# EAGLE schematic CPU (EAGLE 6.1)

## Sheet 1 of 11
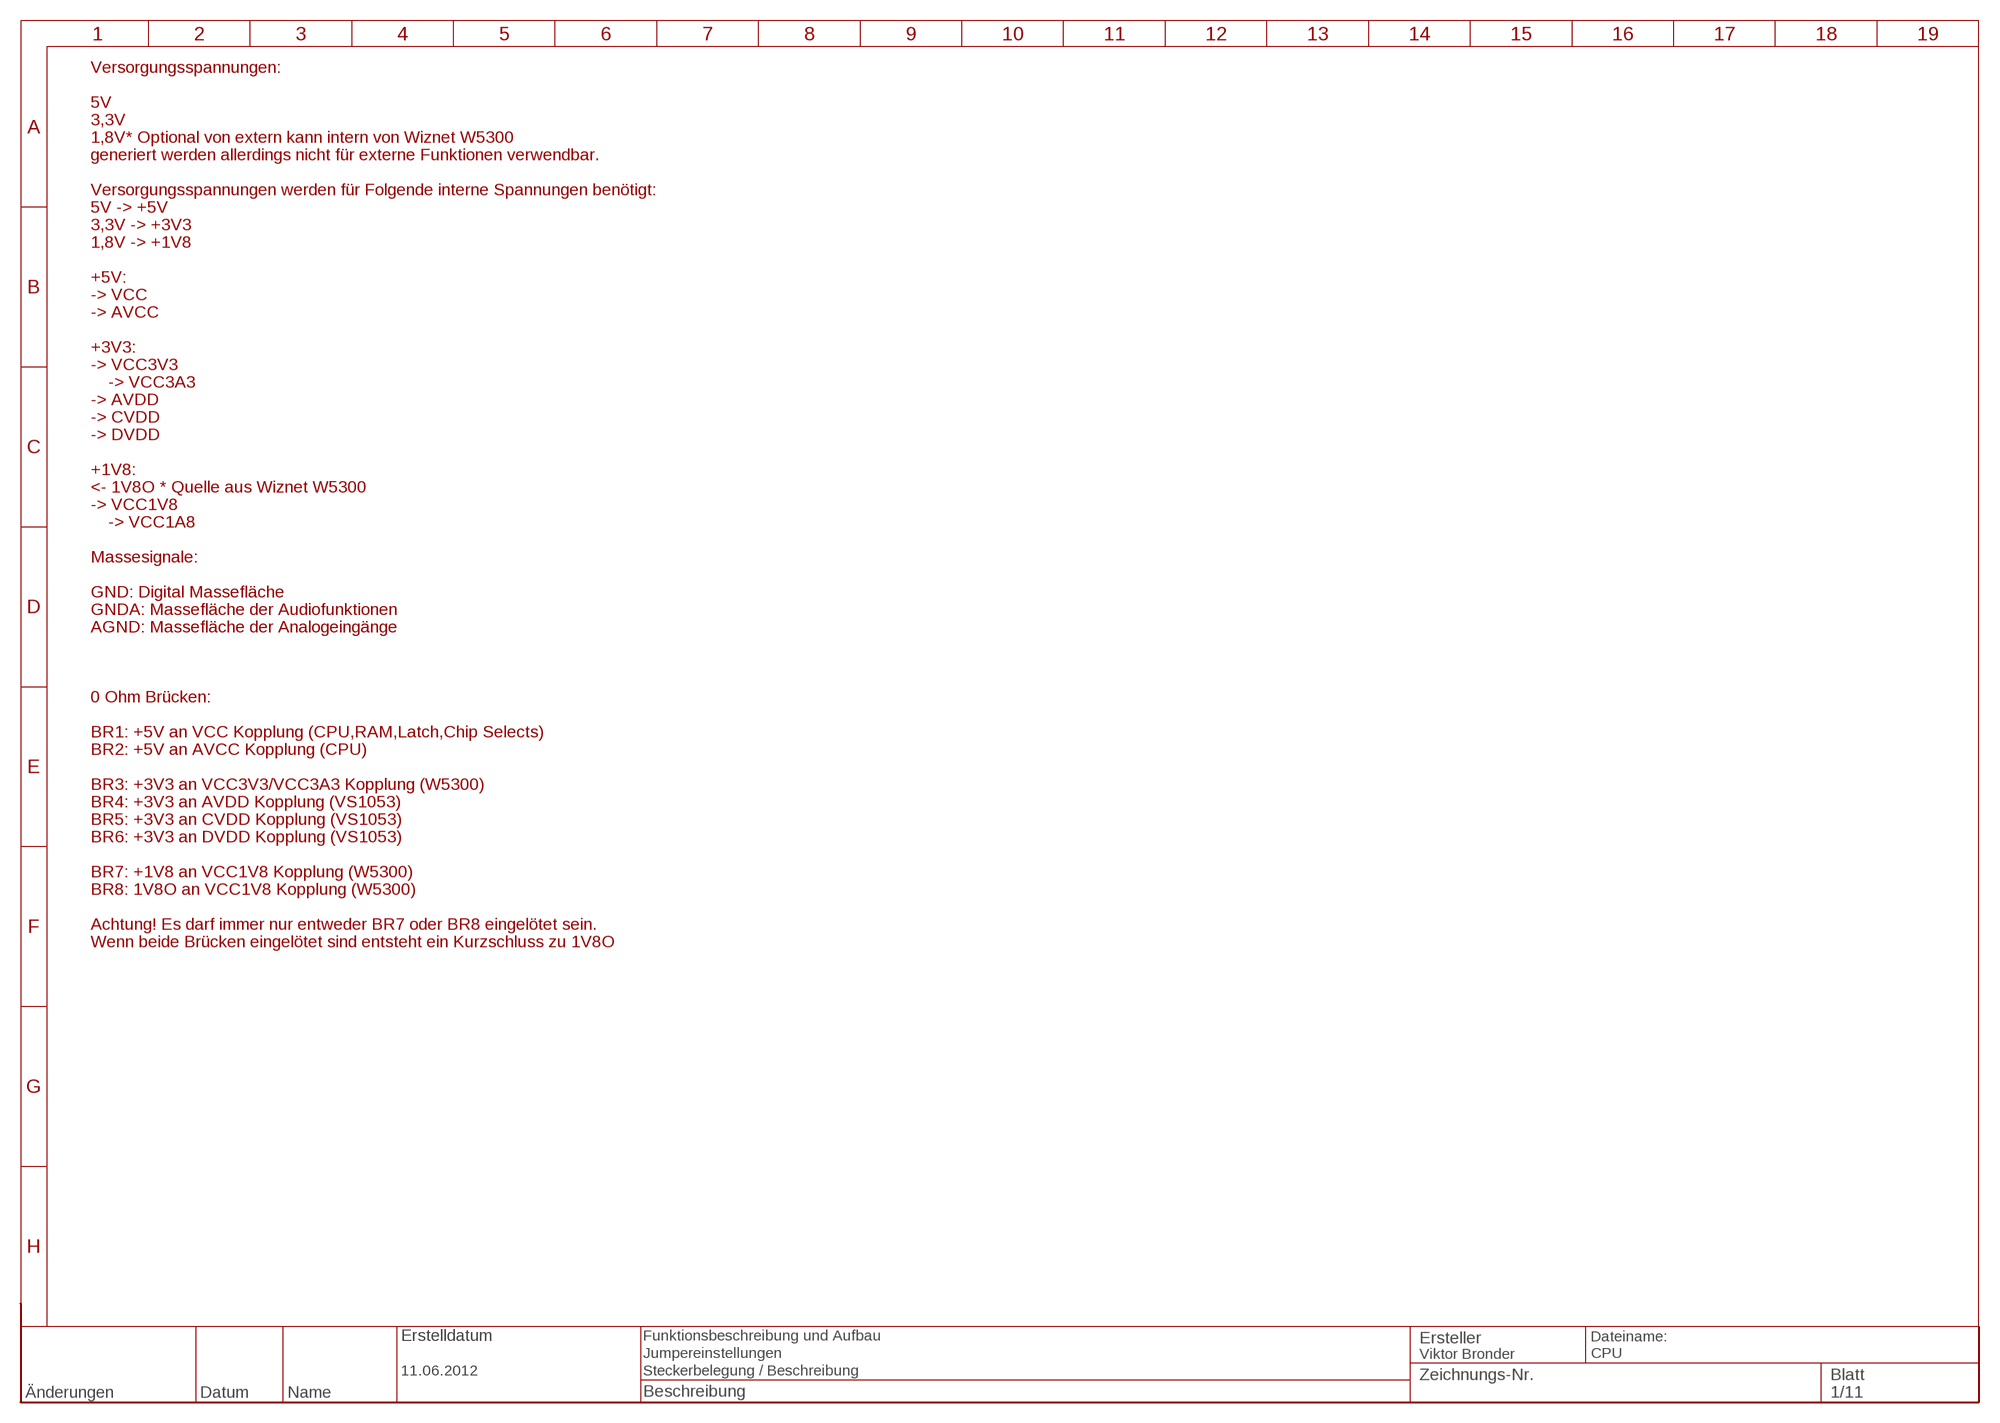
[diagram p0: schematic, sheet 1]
RAHMEN1 (RAHMEN_A4_8Z-19S): BESCHREIBUNG1: Funktionsbeschreibung und Aufbau; BESCHREIBUNG2: Jumpereinstellungen; BESCHREIBUNG3: Steckerbelegung / Beschreibung; ERSTELLDATUM: 11.06.2012; ERSTELLER: Viktor Bronder

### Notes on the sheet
- Versorgungsspannungen:
- 5V
- 3,3V
- 1,8V* Optional von extern kann intern von Wiznet W5300
- generiert werden allerdings nicht für externe Funktionen verwendbar.
- Versorgungsspannungen werden für Folgende interne Spannungen benötigt:
- 5V -> +5V
- 3,3V -> +3V3
- 1,8V -> +1V8
- +5V:
- -> VCC
- -> AVCC
- +3V3:
- -> VCC3V3
- -> VCC3A3
- -> AVDD
- -> CVDD
- -> DVDD
- +1V8:
- <- 1V8O * Quelle aus Wiznet W5300
- -> VCC1V8
- -> VCC1A8
- Massesignale:
- GND: Digital Massefläche
- GNDA: Massefläche der Audiofunktionen
- AGND: Massefläche der Analogeingänge
- 0 Ohm Brücken:
- BR1: +5V an VCC Kopplung (CPU,RAM,Latch,Chip Selects)
- BR2: +5V an AVCC Kopplung (CPU)
- BR3: +3V3 an VCC3V3/VCC3A3 Kopplung (W5300)
- BR4: +3V3 an AVDD Kopplung (VS1053)
- BR5: +3V3 an CVDD Kopplung (VS1053)
- BR6: +3V3 an DVDD Kopplung (VS1053)
- BR7: +1V8 an VCC1V8 Kopplung (W5300)
- BR8: 1V8O an VCC1V8 Kopplung (W5300)
- Achtung! Es darf immer nur entweder BR7 oder BR8 eingelötet sein.
- Wenn beide Brücken eingelötet sind entsteht ein Kurzschluss zu 1V8O

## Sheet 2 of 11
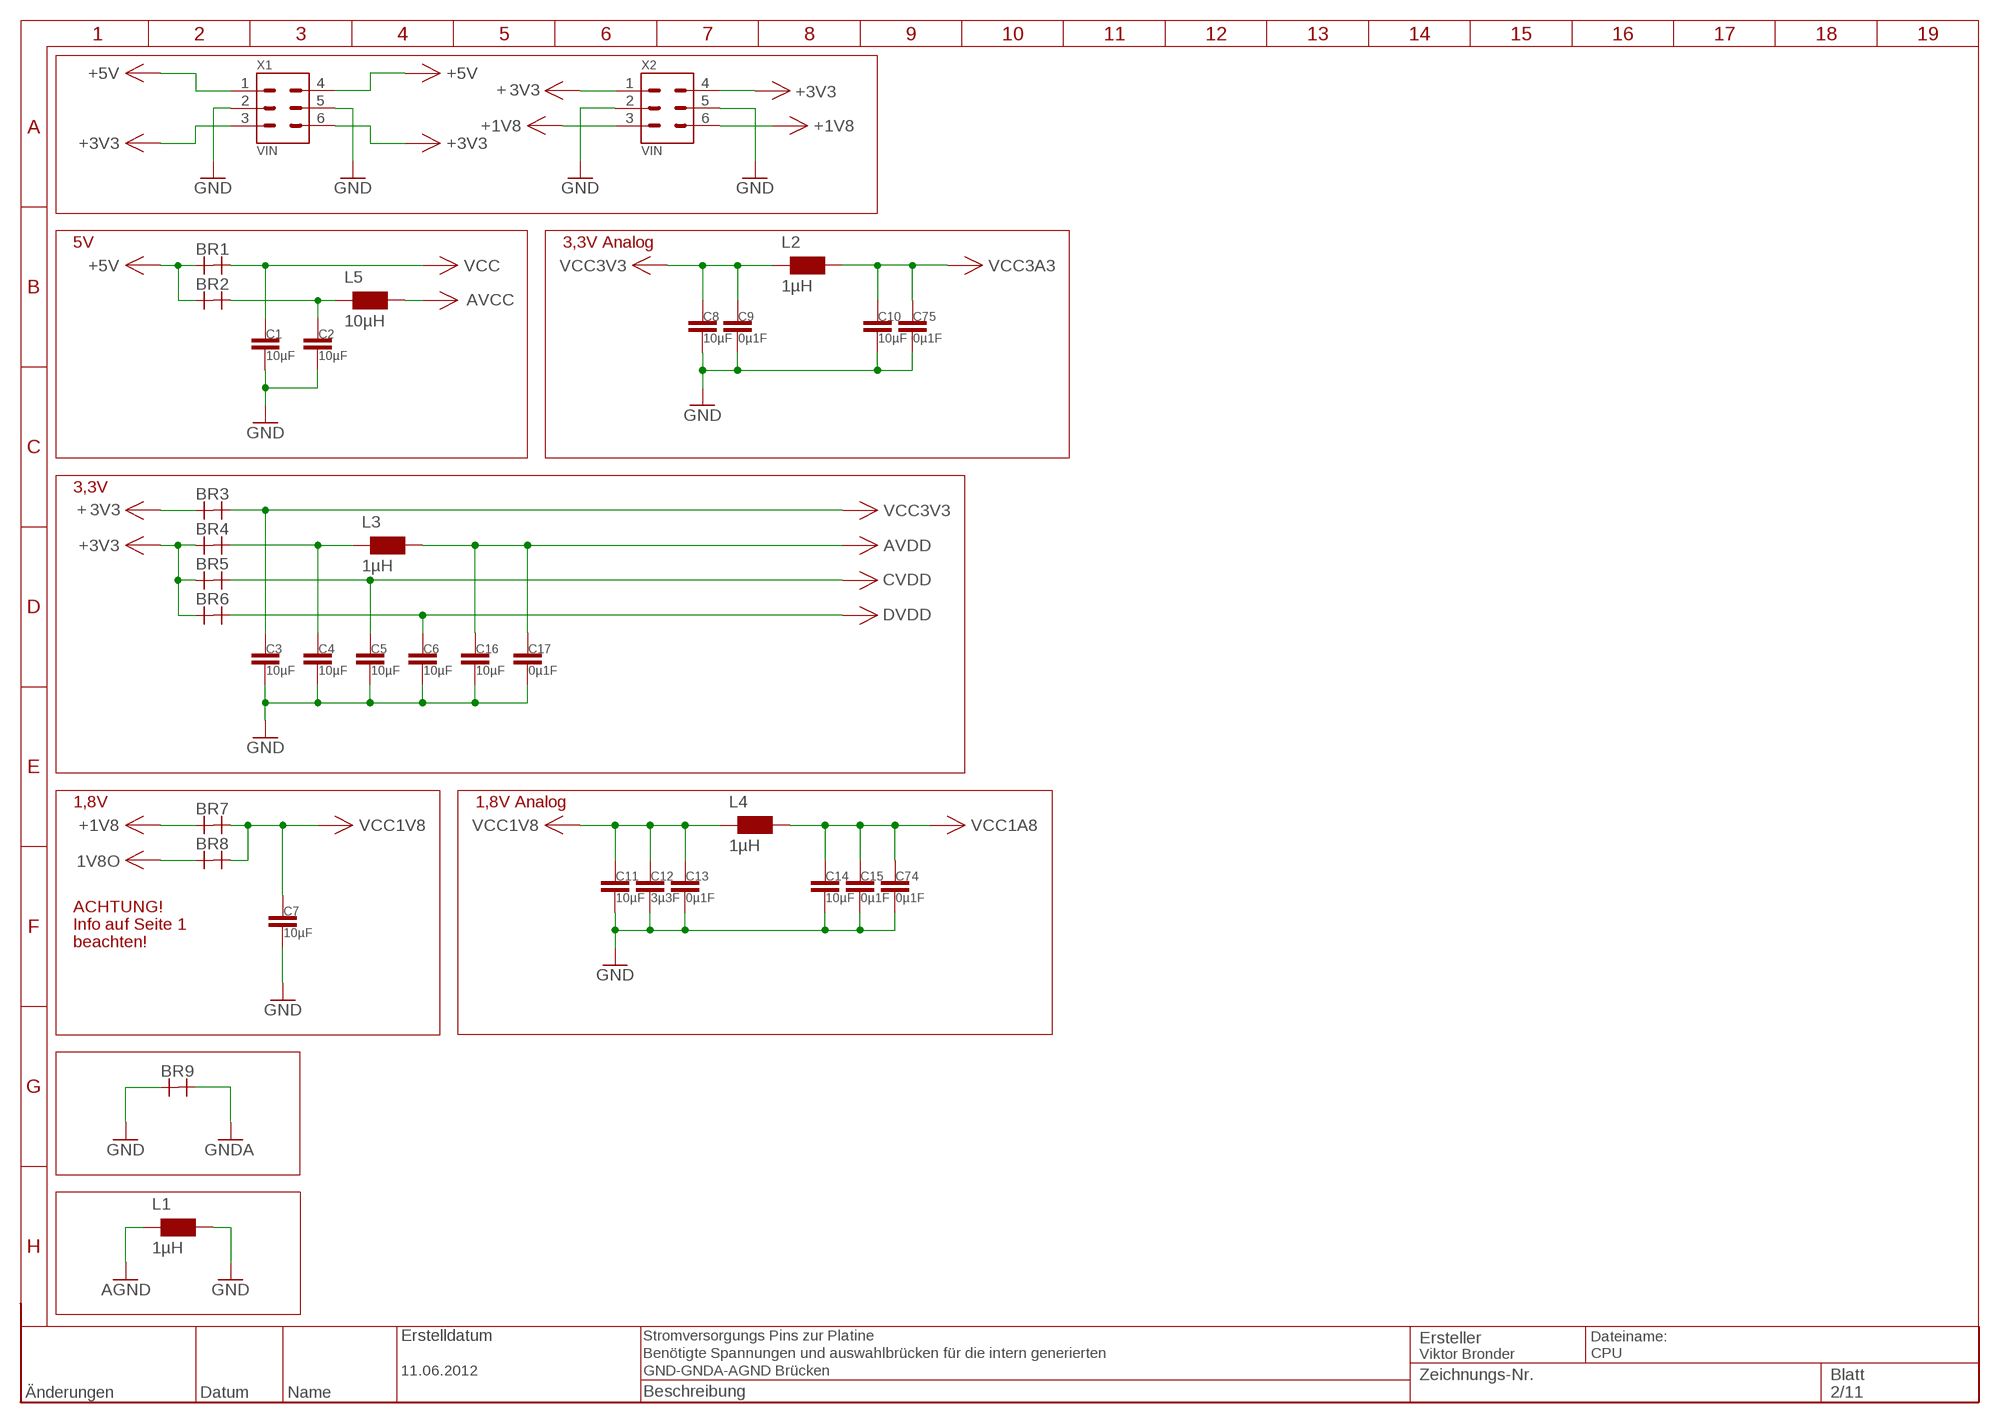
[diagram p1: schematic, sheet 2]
RAHMEN2 (RAHMEN_A4_8Z-19S): BESCHREIBUNG1: Stromversorgungs Pins zur Platine; BESCHREIBUNG2: Benötigte Spannungen und auswahlbrücken für die intern generierten; BESCHREIBUNG3: GND-GNDA-AGND Brücken; ERSTELLDATUM: 11.06.2012; ERSTELLER: Viktor Bronder

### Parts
BR1  0-OHM-BRÜCKE  [0-OHM-BRÜCKE]
BR2  0-OHM-BRÜCKE  [0-OHM-BRÜCKE]
BR3  0-OHM-BRÜCKE  [0-OHM-BRÜCKE]
BR4  0-OHM-BRÜCKE  [0-OHM-BRÜCKE]
BR5  0-OHM-BRÜCKE  [0-OHM-BRÜCKE]
BR6  0-OHM-BRÜCKE  [0-OHM-BRÜCKE]
BR7  0-OHM-BRÜCKE  [0-OHM-BRÜCKE]
BR8  0-OHM-BRÜCKE  [0-OHM-BRÜCKE]
BR9  0-OHM-BRÜCKE  [0-OHM-BRÜCKE]
C1  10µF  C-SMD  [0805]
C2  10µF  C-SMD  [0805]
C3  10µF  C-SMD  [0805]
C4  10µF  C-SMD  [0805]
C5  10µF  C-SMD  [0805]
C6  10µF  C-SMD  [0805]
C7  10µF  C-SMD  [0805]
C8  10µF  C-SMD  [0805]
C9  0µ1F  C-SMD0603  [0603]
C10  10µF  C-SMD  [0805]
C11  10µF  C-SMD  [0805]
C12  3µ3F  C-SMD0603  [0603]
C13  0µ1F  C-SMD0603  [0603]
C14  10µF  C-SMD  [0805]
C15  0µ1F  C-SMD0603  [0603]
C16  10µF  C-SMD  [0805]
C17  0µ1F  C-SMD0603  [0603]
C74  0µ1F  C-SMD0603  [0603]
C75  0µ1F  C-SMD0603  [0603]
L1  1µH  WE-CBF_0805  [0805]
L2  1µH  WE-CBF_0805  [0805]
L3  1µH  WE-CBF_0805  [0805]
L4  1µH  WE-CBF_0805  [0805]
L5  10µH  WE-CBF_0805  [0805]
X1  VIN  STIFTLEISTE-6PIN  [STIFTLEISTE-2X3PIN]
X2  VIN  STIFTLEISTE-6PIN  [STIFTLEISTE-2X3PIN]

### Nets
1V8O: BR8.1 ; also sheet 5
3V3: BR3.1 X2.1 X2.4
+1V8: BR7.1 X2.3 X2.6
+3V3: BR4.1 BR5.1 BR6.1 X1.3 X1.6
+5V: BR1.1 BR2.1 X1.1 X1.4
AGND: L1.1 ; also sheet 3,7
AVCC: L5.2 ; also sheet 3,10
AVDD: C16.1 C17.1 L3.2 ; also sheet 3,7
CVDD: BR5.2 C5.1 ; also sheet 3
DVDD: BR6.2 C6.1 ; also sheet 3,7
GND: BR9.1 C1.2 C2.2 C3.2 C4.2 C5.2 C6.2 C7.2 C8.2 C9.2 C10.2 C11.2 C12.2 C13.2 C14.2 C15.2 C16.2 C17.2 C74.2 C75.2 L1.2 X1.2 X1.5 X2.2 X2.5 ; also sheet 3,4,5,7,10
GNDA: BR9.2 ; also sheet 5,10
N$1: BR4.2 C4.1 L3.1
N$2: BR2.2 C2.1 L5.1
VCC: BR1.2 C1.1 ; also sheet 3,10
VCC1A8: C14.1 C15.1 C74.1 L4.2 ; also sheet 5
VCC1V8: BR7.2 BR8.2 C7.1 C11.1 C12.1 C13.1 L4.1 ; also sheet 3,5
VCC3A3: C10.1 C75.1 L2.2 ; also sheet 5
VCC3V3: BR3.2 C3.1 C8.1 C9.1 L2.1 ; also sheet 3,5,10

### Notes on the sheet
- + | +
- 5V | 3,3V Analog
- 3,3V
- +
- 1,8V | 1,8V Analog
- ACHTUNG!
- Info auf Seite 1
- beachten!

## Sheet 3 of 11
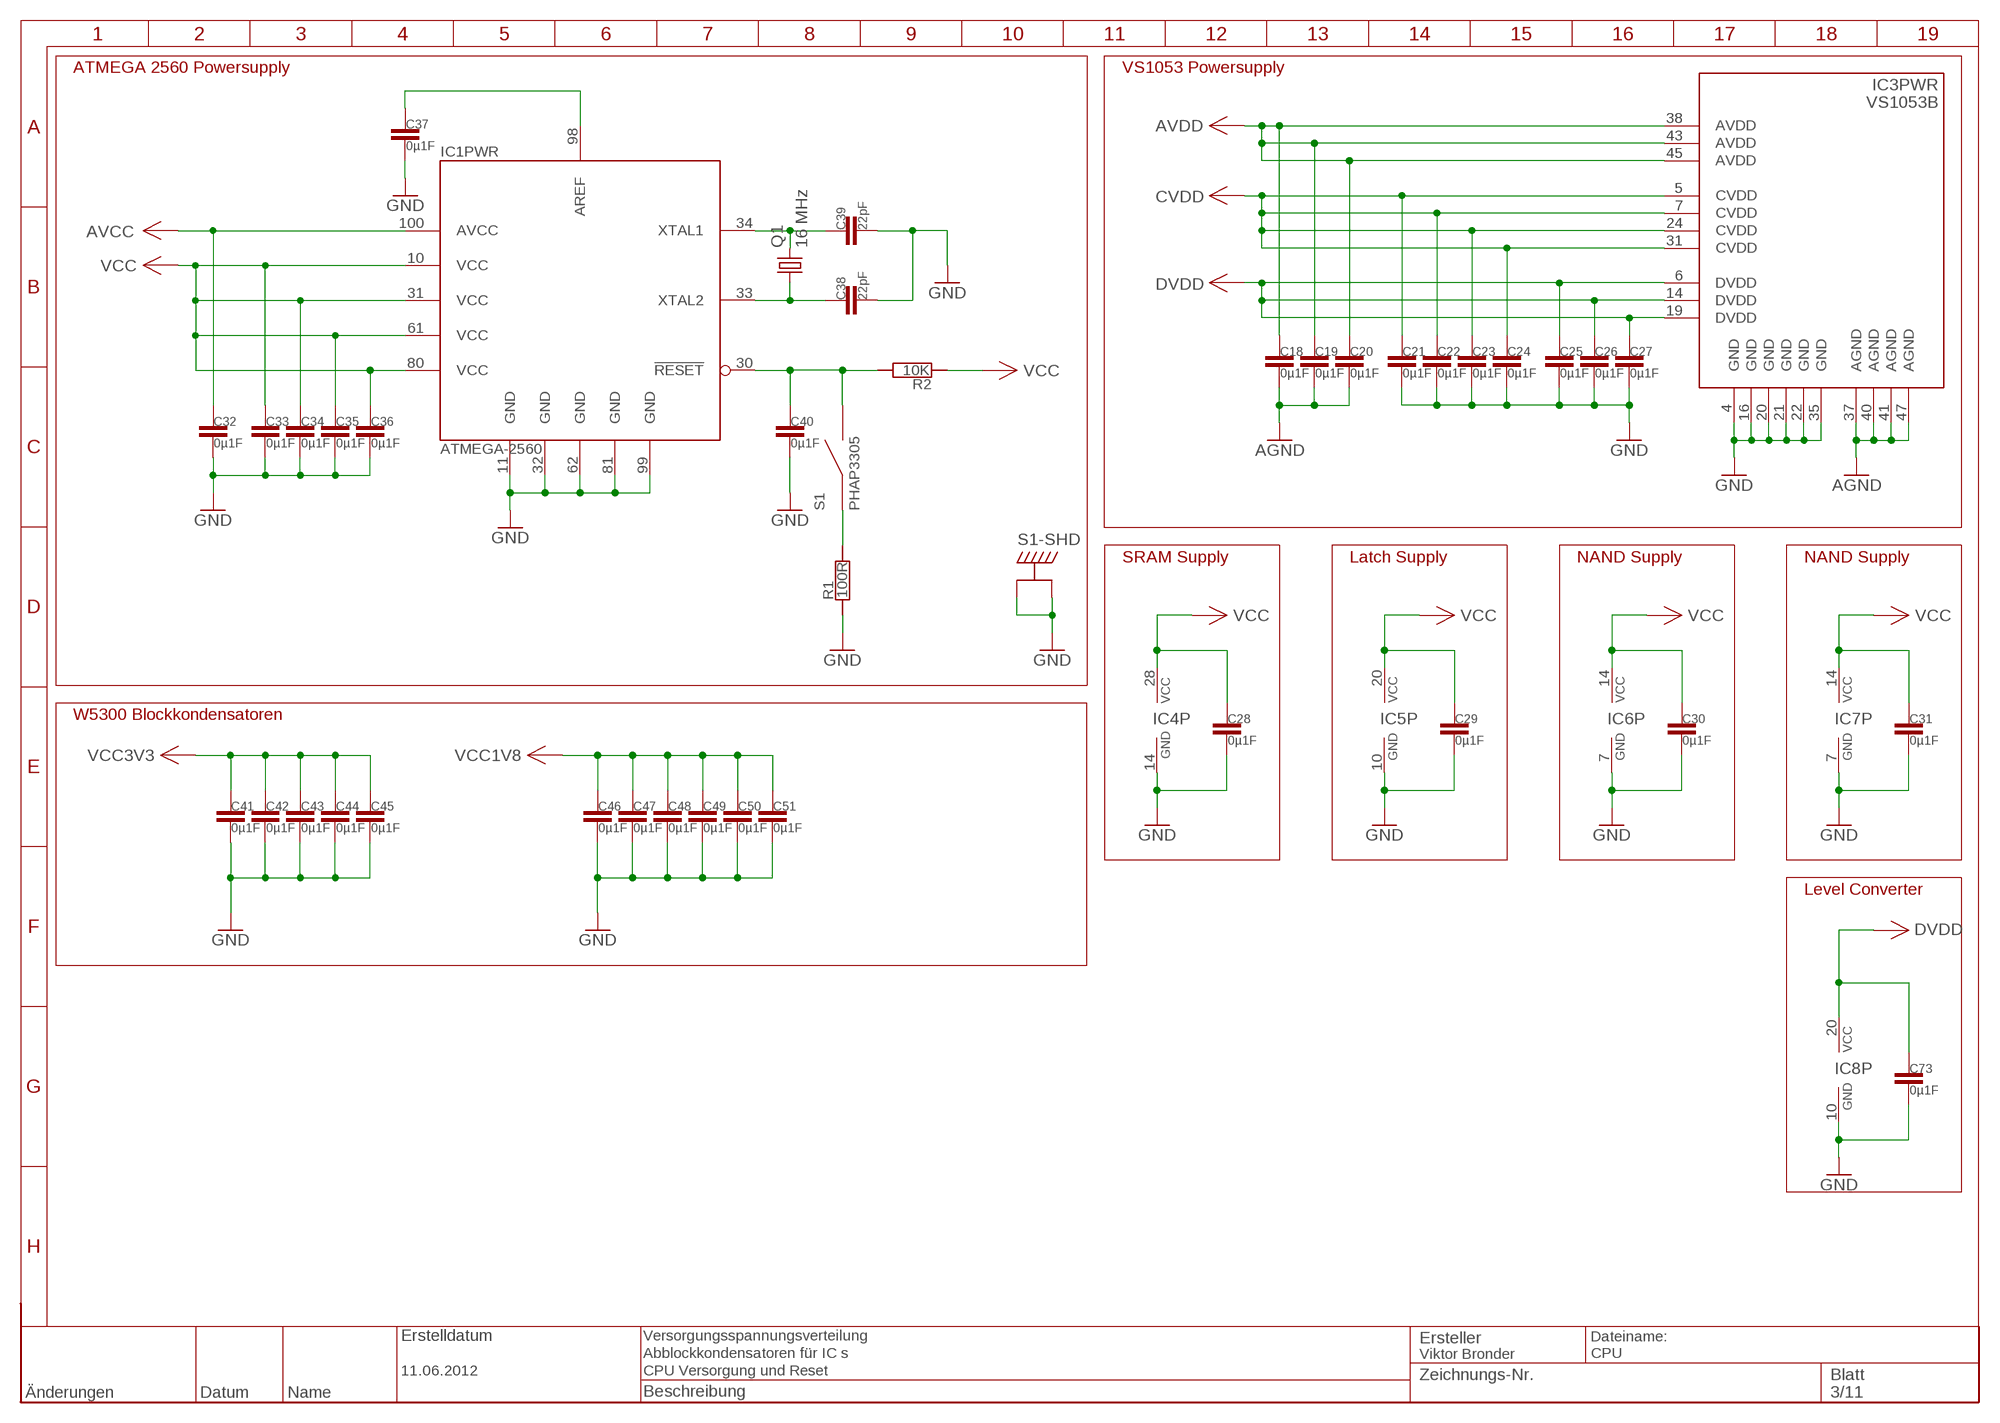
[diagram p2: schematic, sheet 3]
RAHMEN3 (RAHMEN_A4_8Z-19S): BESCHREIBUNG1: Versorgungsspannungsverteilung; BESCHREIBUNG2: Abblockkondensatoren für IC s; BESCHREIBUNG3: CPU Versorgung und Reset; ERSTELLDATUM: 11.06.2012; ERSTELLER: Viktor Bronder

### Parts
C18  0µ1F  C-SMD0603  [0603]
C19  0µ1F  C-SMD0603  [0603]
C20  0µ1F  C-SMD0603  [0603]
C21  0µ1F  C-SMD0603  [0603]
C22  0µ1F  C-SMD0603  [0603]
C23  0µ1F  C-SMD0603  [0603]
C24  0µ1F  C-SMD0603  [0603]
C25  0µ1F  C-SMD0603  [0603]
C26  0µ1F  C-SMD0603  [0603]
C27  0µ1F  C-SMD0603  [0603]
C28  0µ1F  C-SMD0603  [0603]
C29  0µ1F  C-SMD0603  [0603]
C30  0µ1F  C-SMD0603  [0603]
C31  0µ1F  C-SMD0603  [0603]
C32  0µ1F  C-SMD0603  [0603]
C33  0µ1F  C-SMD0603  [0603]
C34  0µ1F  C-SMD0603  [0603]
C35  0µ1F  C-SMD0603  [0603]
C36  0µ1F  C-SMD0603  [0603]
C37  0µ1F  C-SMD0603  [0603]
C38  22pF  C-SMD0603  [0603]
C39  22pF  C-SMD0603  [0603]
C40  0µ1F  C-SMD0603  [0603]
C41  0µ1F  C-SMD0603  [0603]
C42  0µ1F  C-SMD0603  [0603]
C43  0µ1F  C-SMD0603  [0603]
C44  0µ1F  C-SMD0603  [0603]
C45  0µ1F  C-SMD0603  [0603]
C46  0µ1F  C-SMD0603  [0603]
C47  0µ1F  C-SMD0603  [0603]
C48  0µ1F  C-SMD0603  [0603]
C49  0µ1F  C-SMD0603  [0603]
C50  0µ1F  C-SMD0603  [0603]
C51  0µ1F  C-SMD0603  [0603]
C73  0µ1F  C-SMD0603  [0603]
IC1  ATMEGA-2560  [TQFP100]
IC3  VS1053B  VLSI-VS1053B  [TQFP48]
IC4  62256-70M  TC55257DF  [SOP28X]
IC5  74VHC573D  74AC573D  [SO20W]
IC6  7400  74HCT00D  [SO14]
IC7  7400  74HCT00D  [SO14]
IC8  74HCT244DW  [SO20W]
Q1  16 MHz  CRYSTALHC49U-V  [HC49U-V]
R1  100R  R-SMD0603  [0603]
R2  10K  R-SMD0603  [0603]
S1  PHAP3305  [PHAP3305]

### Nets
AGND: C18.2 C19.2 C20.2 IC3.37(AGND) IC3.40(AGND) IC3.41(AGND) IC3.47(AGND) ; also sheet 2,7
AVCC: C32.1 IC1.100(PWR:AVCC) ; also sheet 2,10
AVDD: C18.1 C19.1 C20.1 IC3.38(AVDD) IC3.43(AVDD) IC3.45(AVDD) ; also sheet 2,7
CVDD: C21.1 C22.1 C23.1 C24.1 IC3.5(CVDD) IC3.7(CVDD) IC3.24(CVDD) IC3.31(CVDD) ; also sheet 2
DVDD: C25.1 C26.1 C27.1 C73.1 IC3.6(DVDD) IC3.14(DVDD) IC3.19(DVDD) IC8.20(P:VCC) ; also sheet 2,7
GND: C21.2 C22.2 C23.2 C24.2 C25.2 C26.2 C27.2 C28.2 C29.2 C30.2 C31.2 C32.2 C33.2 C34.2 C35.2 C36.2 C37.2 C38.2 C39.2 C40.2 C41.2 C42.2 C43.2 C44.2 C45.2 C46.2 C47.2 C48.2 C49.2 C50.2 C51.2 C73.2 IC1.11(PWR:GND) IC1.32(PWR:GND) IC1.62(PWR:GND) IC1.81(PWR:GND) IC1.99(PWR:GND) IC3.4(GND) IC3.16(GND) IC3.20(GND) IC3.21(GND) IC3.22(GND) IC3.35(GND) IC4.14(GND) IC5.10(GND) IC6.7(P:GND) IC7.7(P:GND) IC8.10(P:GND) R1.1 S1.SHD@0(SHD) S1.SHD@1(SHD) ; also sheet 2,4,5,7,10
N$3: C39.1 IC1.34(PWR:XTAL1) Q1.2
N$4: C38.1 IC1.33(PWR:XTAL2) Q1.1
N$5: C37.1 IC1.98(PWR:AREF)
N$6: C40.1 IC1.30(PWR:!RESET) R2.2 S1.2
N$7: R1.2 S1.1
VCC: C28.1 C29.1 C30.1 C31.1 C33.1 C34.1 C35.1 C36.1 IC1.10(PWR:VCC) IC1.31(PWR:VCC) IC1.61(PWR:VCC) IC1.80(PWR:VCC) IC4.28(VCC) IC5.20(VCC) IC6.14(P:VCC) IC7.14(P:VCC) R2.1 ; also sheet 2,10
VCC1V8: C46.1 C47.1 C48.1 C49.1 C50.1 C51.1 ; also sheet 2,5
VCC3V3: C41.1 C42.1 C43.1 C44.1 C45.1 ; also sheet 2,5,10

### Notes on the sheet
- ATMEGA 2560 Powersupply | VS1053 Powersupply
- SRAM Supply | Latch Supply | NAND Supply | NAND Supply
- W5300 Blockkondensatoren
- Level Converter

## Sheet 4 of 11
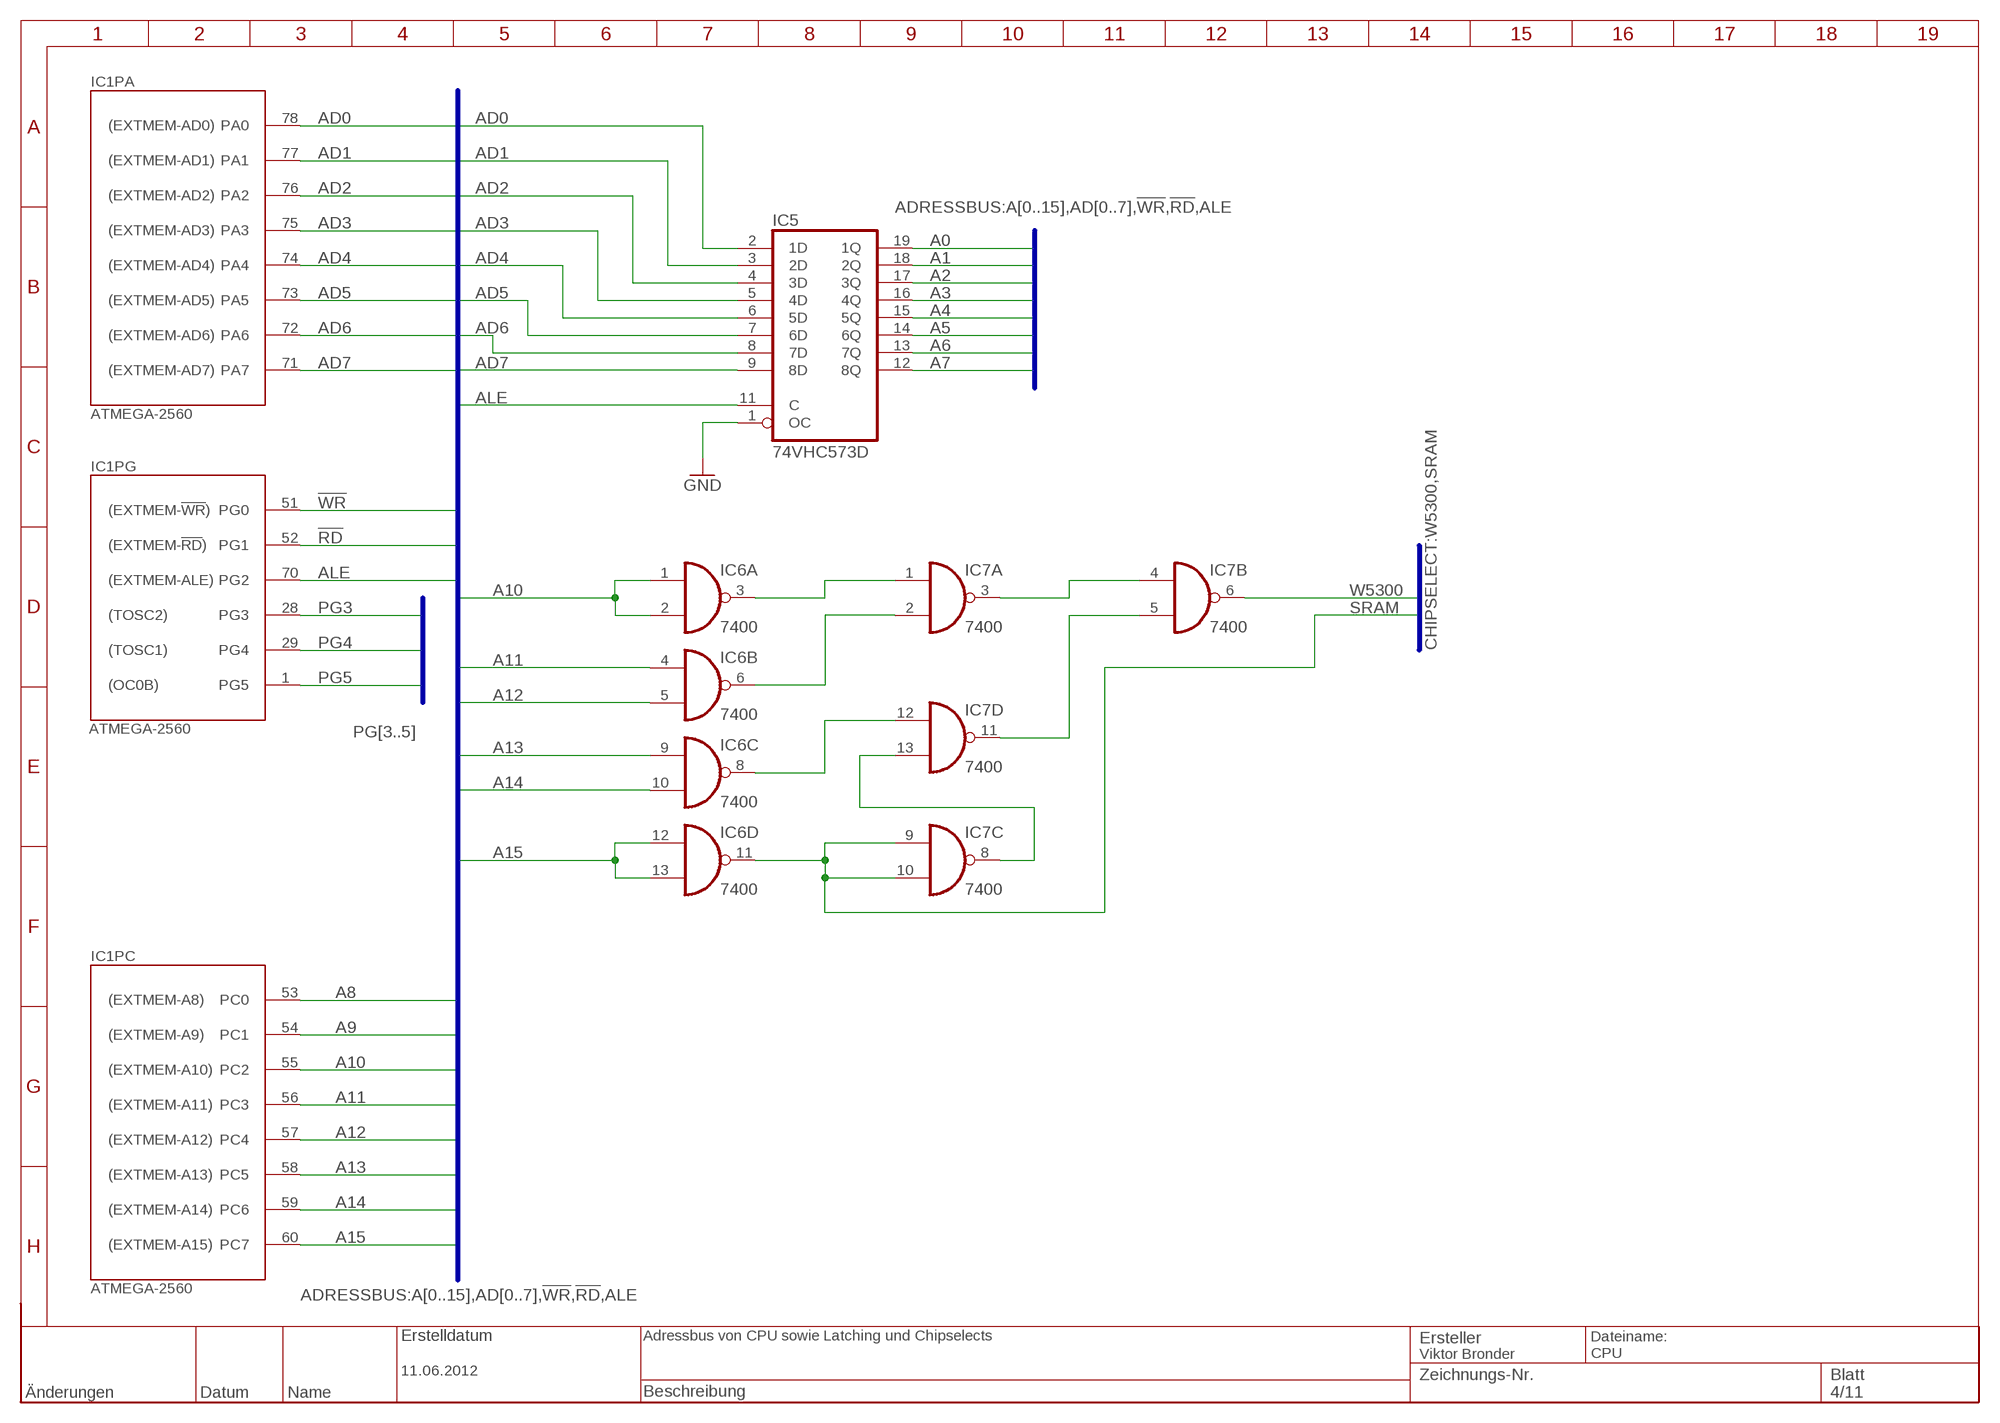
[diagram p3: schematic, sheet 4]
RAHMEN4 (RAHMEN_A4_8Z-19S): BESCHREIBUNG1: Adressbus von CPU sowie Latching und Chipselects; ERSTELLDATUM: 11.06.2012; ERSTELLER: Viktor Bronder

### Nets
!RD: IC1.52(PG:PG1) ; also sheet 5,6
!WR: IC1.51(PG:PG0) ; also sheet 5,6
A0: IC5.19(1Q) ; also sheet 5,6
A1: IC5.18(2Q) ; also sheet 5,6
A2: IC5.17(3Q) ; also sheet 5,6
A3: IC5.16(4Q) ; also sheet 5,6
A4: IC5.15(5Q) ; also sheet 5,6
A5: IC5.14(6Q) ; also sheet 5,6
A6: IC5.13(7Q) ; also sheet 5,6
A7: IC5.12(8Q) ; also sheet 5,6
A8: IC1.53(PC:PC0) ; also sheet 5,6
A9: IC1.54(PC:PC1) ; also sheet 5,6
A10: IC1.55(PC:PC2) IC6.1(A:I0) IC6.2(A:I1) ; also sheet 6
A11: IC1.56(PC:PC3) IC6.4(B:I0) ; also sheet 6
A12: IC1.57(PC:PC4) IC6.5(B:I1) ; also sheet 6
A13: IC1.58(PC:PC5) IC6.9(C:I0) ; also sheet 6
A14: IC1.59(PC:PC6) IC6.10(C:I1) ; also sheet 6
A15: IC1.60(PC:PC7) IC6.12(D:I0) IC6.13(D:I1)
AD0: IC1.78(PA:PA0) IC5.2(1D) ; also sheet 5,6
AD1: IC1.77(PA:PA1) IC5.3(2D) ; also sheet 5,6
AD2: IC1.76(PA:PA2) IC5.4(3D) ; also sheet 5,6
AD3: IC1.75(PA:PA3) IC5.5(4D) ; also sheet 5,6
AD4: IC1.74(PA:PA4) IC5.6(5D) ; also sheet 5,6
AD5: IC1.73(PA:PA5) IC5.7(6D) ; also sheet 5,6
AD6: IC1.72(PA:PA6) IC5.8(7D) ; also sheet 5,6
AD7: IC1.71(PA:PA7) IC5.9(8D) ; also sheet 5,6
ALE: IC1.70(PG:PG2) IC5.11(C)
GND: IC5.1(OC) ; also sheet 2,3,5,7,10
N$8: IC6.3(A:O) IC7.1(A:I0)
N$9: IC6.6(B:O) IC7.2(A:I1)
N$10: IC7.3(A:O) IC7.4(B:I0)
N$11: IC6.8(C:O) IC7.12(D:I0)
N$12: IC7.8(C:O) IC7.13(D:I1)
N$13: IC7.5(B:I1) IC7.11(D:O)
PG3: IC1.28(PG:PG3) ; also sheet 10
PG4: IC1.29(PG:PG4) ; also sheet 10
PG5: IC1.1(PG:PG5) ; also sheet 10
SRAM: IC6.11(D:O) IC7.9(C:I0) IC7.10(C:I1) ; also sheet 6
W5300: IC7.6(B:O) ; also sheet 5

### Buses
ADRESSBUS:A[0..15],AD[0..7],!WR,!RD,ALE
CHIPSELECT:W5300,SRAM
PG[3..5]

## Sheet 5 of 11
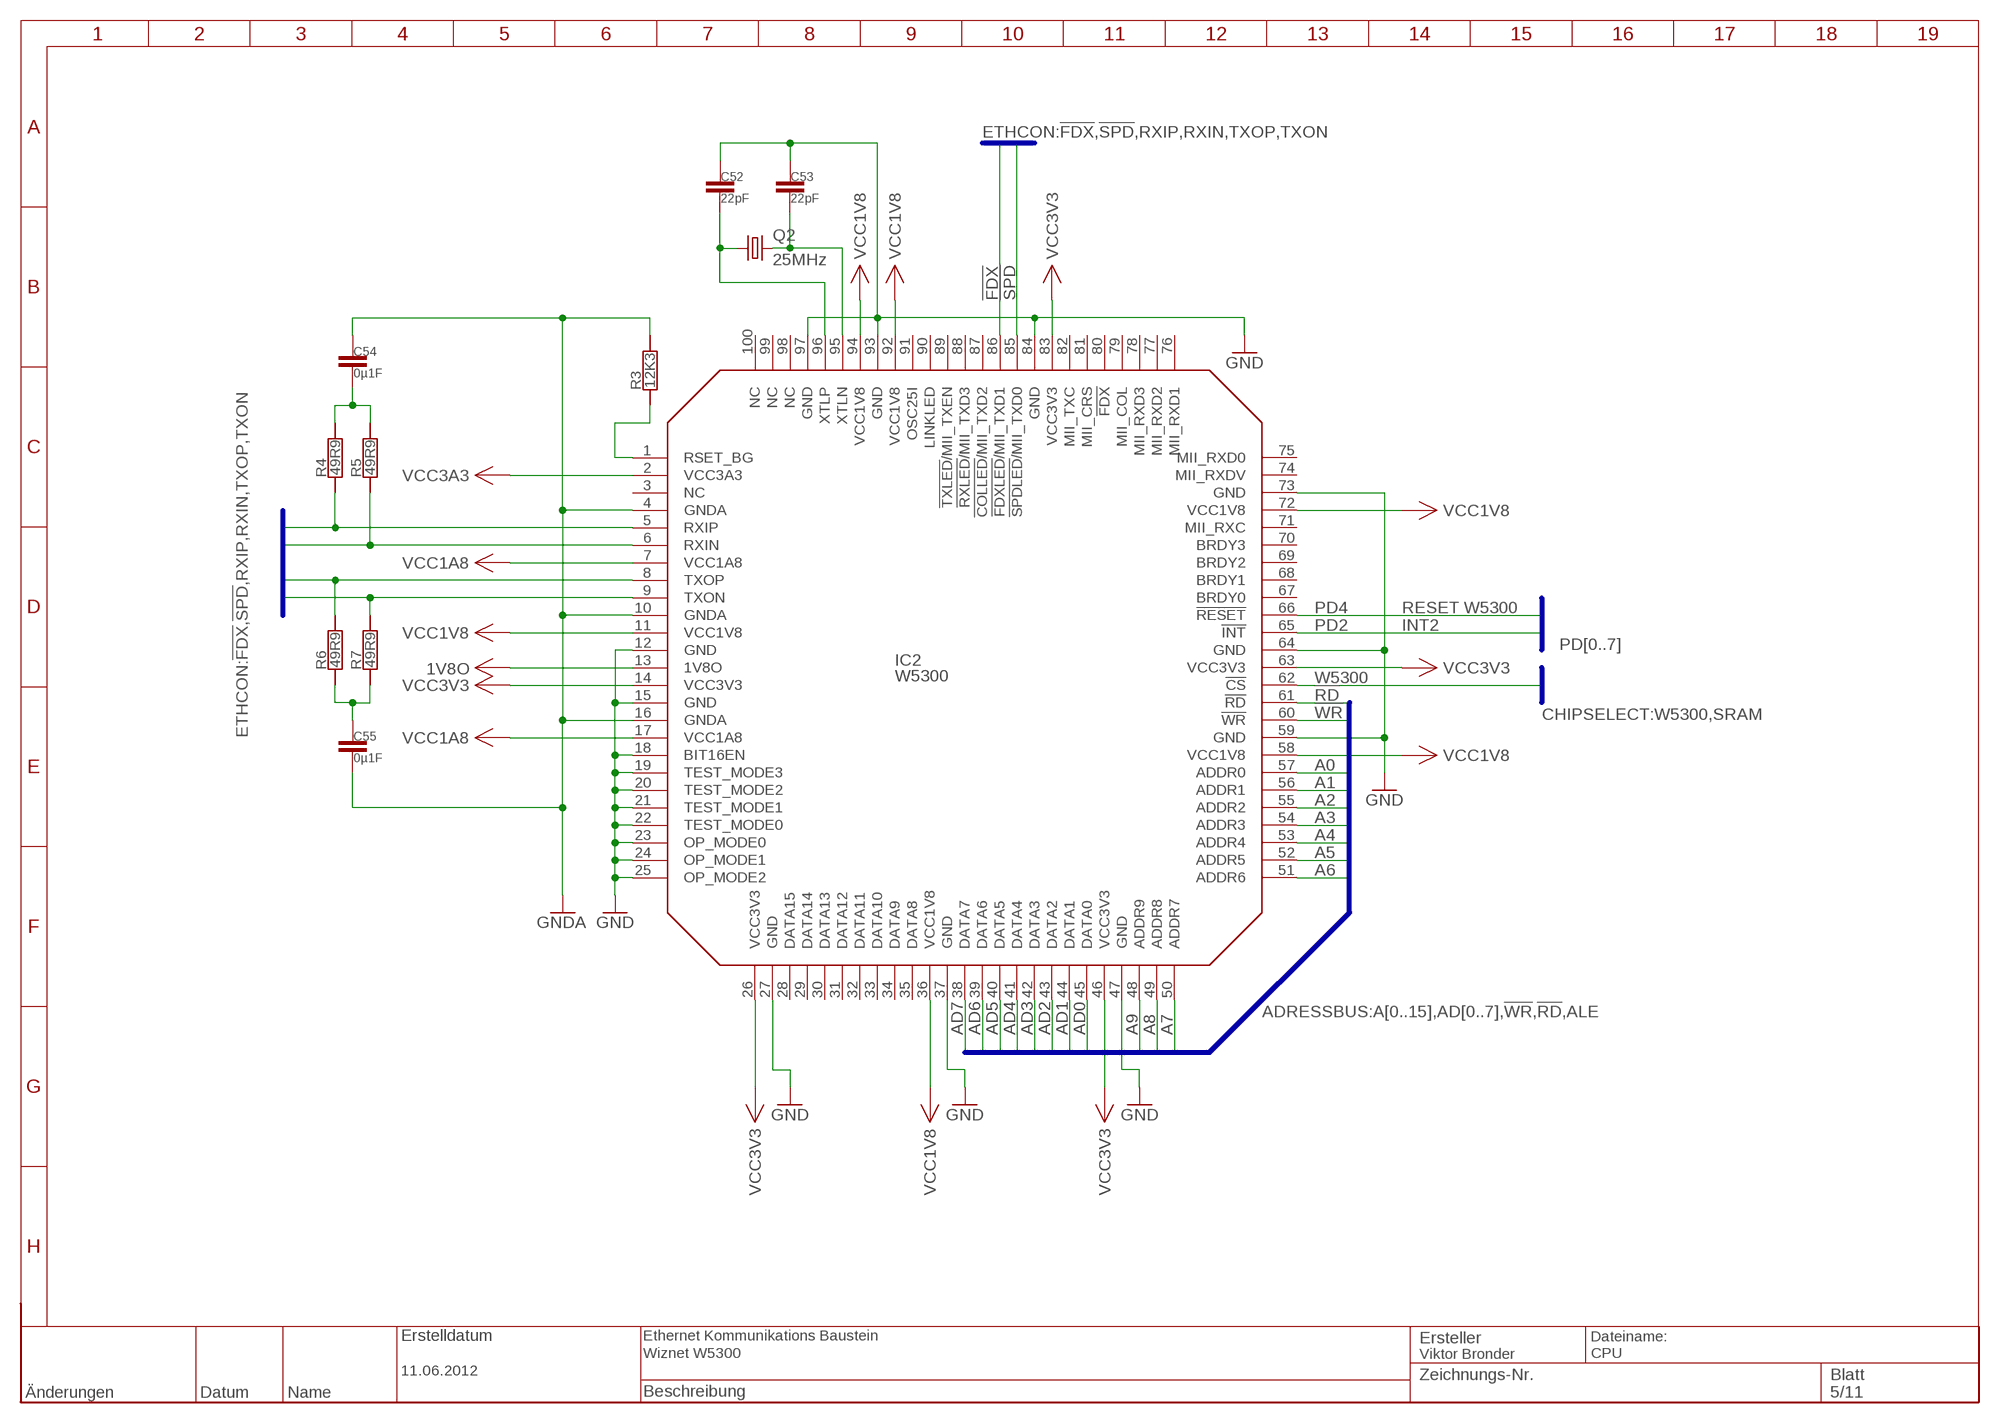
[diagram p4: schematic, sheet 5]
RAHMEN5 (RAHMEN_A4_8Z-19S): BESCHREIBUNG1: Ethernet Kommunikations Baustein; BESCHREIBUNG2: Wiznet W5300; ERSTELLDATUM: 11.06.2012; ERSTELLER: Viktor Bronder

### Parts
C52  22pF  C-SMD0603  [0603]
C53  22pF  C-SMD0603  [0603]
C54  0µ1F  C-SMD0603  [0603]
C55  0µ1F  C-SMD0603  [0603]
IC2  W5300  WIZNET-W5300  [TQFP100]
Q2  25MHz  CRYSTALHC49U-V  [HC49U-V]
R3  12K3  R-SMD  [0805]
R4  49R9  R-SMD  [0805]
R5  49R9  R-SMD  [0805]
R6  49R9  R-SMD  [0805]
R7  49R9  R-SMD  [0805]

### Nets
1V8O: IC2.13(1V8O) ; also sheet 2
!FDX: IC2.86(!FDXLED!/MII_TXD1) ; also sheet 10
!RD: IC2.61(!RD) ; also sheet 4,6
!SPD: IC2.85(!SPDLED!/MII_TXD0) ; also sheet 10
!WR: IC2.60(!WR) ; also sheet 4,6
A0: IC2.57(ADDR0) ; also sheet 4,6
A1: IC2.56(ADDR1) ; also sheet 4,6
A2: IC2.55(ADDR2) ; also sheet 4,6
A3: IC2.54(ADDR3) ; also sheet 4,6
A4: IC2.53(ADDR4) ; also sheet 4,6
A5: IC2.52(ADDR5) ; also sheet 4,6
A6: IC2.51(ADDR6) ; also sheet 4,6
A7: IC2.50(ADDR7) ; also sheet 4,6
A8: IC2.49(ADDR8) ; also sheet 4,6
A9: IC2.48(ADDR9) ; also sheet 4,6
AD0: IC2.45(DATA0) ; also sheet 4,6
AD1: IC2.44(DATA1) ; also sheet 4,6
AD2: IC2.43(DATA2) ; also sheet 4,6
AD3: IC2.42(DATA3) ; also sheet 4,6
AD4: IC2.41(DATA4) ; also sheet 4,6
AD5: IC2.40(DATA5) ; also sheet 4,6
AD6: IC2.39(DATA6) ; also sheet 4,6
AD7: IC2.38(DATA7) ; also sheet 4,6
GND: C52.1 C53.1 IC2.12(GND) IC2.15(GND) IC2.18(BIT16EN) IC2.19(TEST_MODE3) IC2.20(TEST_MODE2) IC2.21(TEST_MODE1) IC2.22(TEST_MODE0) IC2.23(OP_MODE0) IC2.24(OP_MODE1) IC2.25(OP_MODE2) IC2.27(GND) IC2.37(GND) IC2.47(GND) IC2.59(GND) IC2.64(GND) IC2.73(GND) IC2.84(GND) IC2.93(GND) IC2.97(GND) ; also sheet 2,3,4,7,10
GNDA: C54.1 C55.2 IC2.4(GNDA) IC2.10(GNDA) IC2.16(GNDA) R3.2 ; also sheet 2,10
N$14: C53.2 IC2.95(XTLN) Q2.2
N$15: C52.2 IC2.96(XTLP) Q2.1
N$16: IC2.1(RSET_BG) R3.1
N$17: C55.1 R6.1 R7.1
N$18: C54.2 R4.2 R5.2
PD2: IC2.65(!INT) ; also sheet 8
PD4: IC2.66(!RESET) ; also sheet 8
RXIN: IC2.6(RXIN) R5.1 ; also sheet 10
RXIP: IC2.5(RXIP) R4.1 ; also sheet 10
TXON: IC2.9(TXON) R7.2 ; also sheet 10
TXOP: IC2.8(TXOP) R6.2 ; also sheet 10
VCC1A8: IC2.7(VCC1A8) IC2.17(VCC1A8) ; also sheet 2
VCC1V8: IC2.11(VCC1V8) IC2.36(VCC1V8) IC2.58(VCC1V8) IC2.72(VCC1V8) IC2.92(VCC1V8) IC2.94(VCC1V8) ; also sheet 2,3
VCC3A3: IC2.2(VCC3A3) ; also sheet 2
VCC3V3: IC2.14(VCC3V3) IC2.26(VCC3V3) IC2.46(VCC3V3) IC2.63(VCC3V3) IC2.83(VCC3V3) ; also sheet 2,3,10
W5300: IC2.62(!CS) ; also sheet 4
Unconnected: IC2.3(NC) IC2.28(DATA15) IC2.29(DATA14) IC2.30(DATA13) IC2.31(DATA12) IC2.32(DATA11) IC2.33(DATA10) IC2.34(DATA9) IC2.35(DATA8) IC2.67(BRDY0) IC2.68(BRDY1) IC2.69(BRDY2) IC2.70(BRDY3) IC2.71(MII_RXC) IC2.74(MII_RXDV) IC2.75(MII_RXD0) IC2.76(MII_RXD1) IC2.77(MII_RXD2) IC2.78(MII_RXD3) IC2.79(MII_COL) IC2.80(!FDX) IC2.81(MII_CRS) IC2.82(MII_TXC) IC2.87(!COLLED!/MII_TXD2) IC2.88(!RXLED!/MII_TXD3) IC2.89(!TXLED!/MII_TXEN) IC2.90(LINKLED) IC2.91(OSC25I) IC2.98(NC) IC2.99(NC) IC2.100(NC)

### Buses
ADRESSBUS:A[0..15],AD[0..7],!WR,!RD,ALE
CHIPSELECT:W5300,SRAM
ETHCON:!FDX,!SPD,RXIP,RXIN,TXOP,TXON
PD[0..7]

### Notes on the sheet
- RESET W5300
- INT2

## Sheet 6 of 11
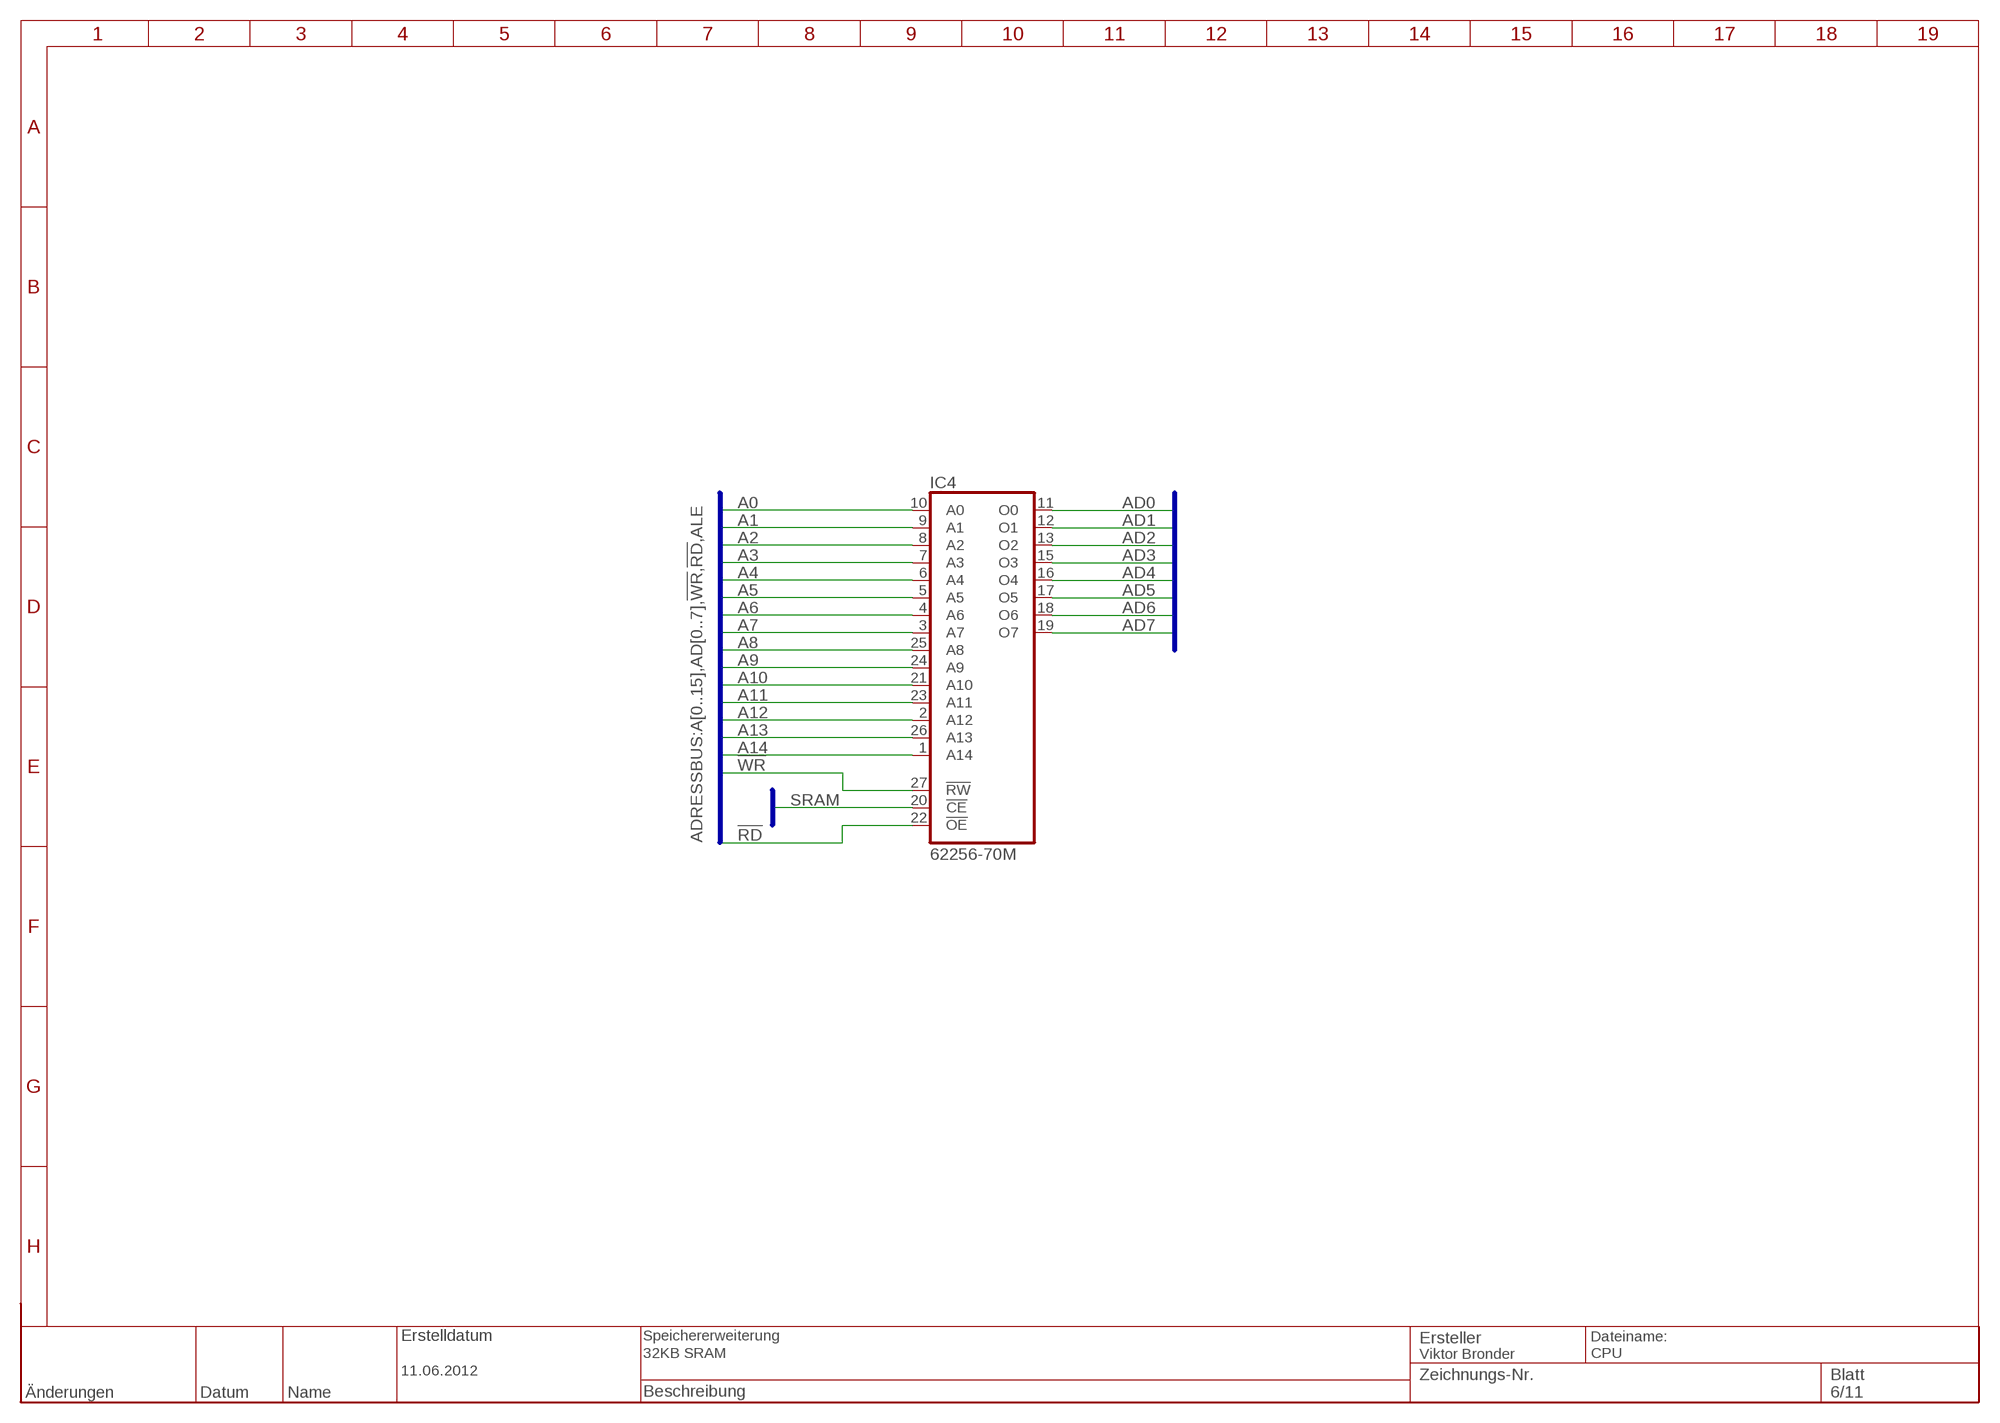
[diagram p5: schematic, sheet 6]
RAHMEN6 (RAHMEN_A4_8Z-19S): BESCHREIBUNG1: Speichererweiterung; BESCHREIBUNG2: 32KB SRAM; ERSTELLDATUM: 11.06.2012; ERSTELLER: Viktor Bronder

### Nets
!RD: IC4.22(!OE) ; also sheet 4,5
!WR: IC4.27(!RW) ; also sheet 4,5
A0: IC4.10(A0) ; also sheet 4,5
A1: IC4.9(A1) ; also sheet 4,5
A2: IC4.8(A2) ; also sheet 4,5
A3: IC4.7(A3) ; also sheet 4,5
A4: IC4.6(A4) ; also sheet 4,5
A5: IC4.5(A5) ; also sheet 4,5
A6: IC4.4(A6) ; also sheet 4,5
A7: IC4.3(A7) ; also sheet 4,5
A8: IC4.25(A8) ; also sheet 4,5
A9: IC4.24(A9) ; also sheet 4,5
A10: IC4.21(A10) ; also sheet 4
A11: IC4.23(A11) ; also sheet 4
A12: IC4.2(A12) ; also sheet 4
A13: IC4.26(A13) ; also sheet 4
A14: IC4.1(A14) ; also sheet 4
AD0: IC4.11(O0) ; also sheet 4,5
AD1: IC4.12(O1) ; also sheet 4,5
AD2: IC4.13(O2) ; also sheet 4,5
AD3: IC4.15(O3) ; also sheet 4,5
AD4: IC4.16(O4) ; also sheet 4,5
AD5: IC4.17(O5) ; also sheet 4,5
AD6: IC4.18(O6) ; also sheet 4,5
AD7: IC4.19(O7) ; also sheet 4,5
SRAM: IC4.20(!CE) ; also sheet 4

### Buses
CHIPSELECT:W5300,SRAM
ADRESSBUS:A[0..15],AD[0..7],!WR,!RD,ALE

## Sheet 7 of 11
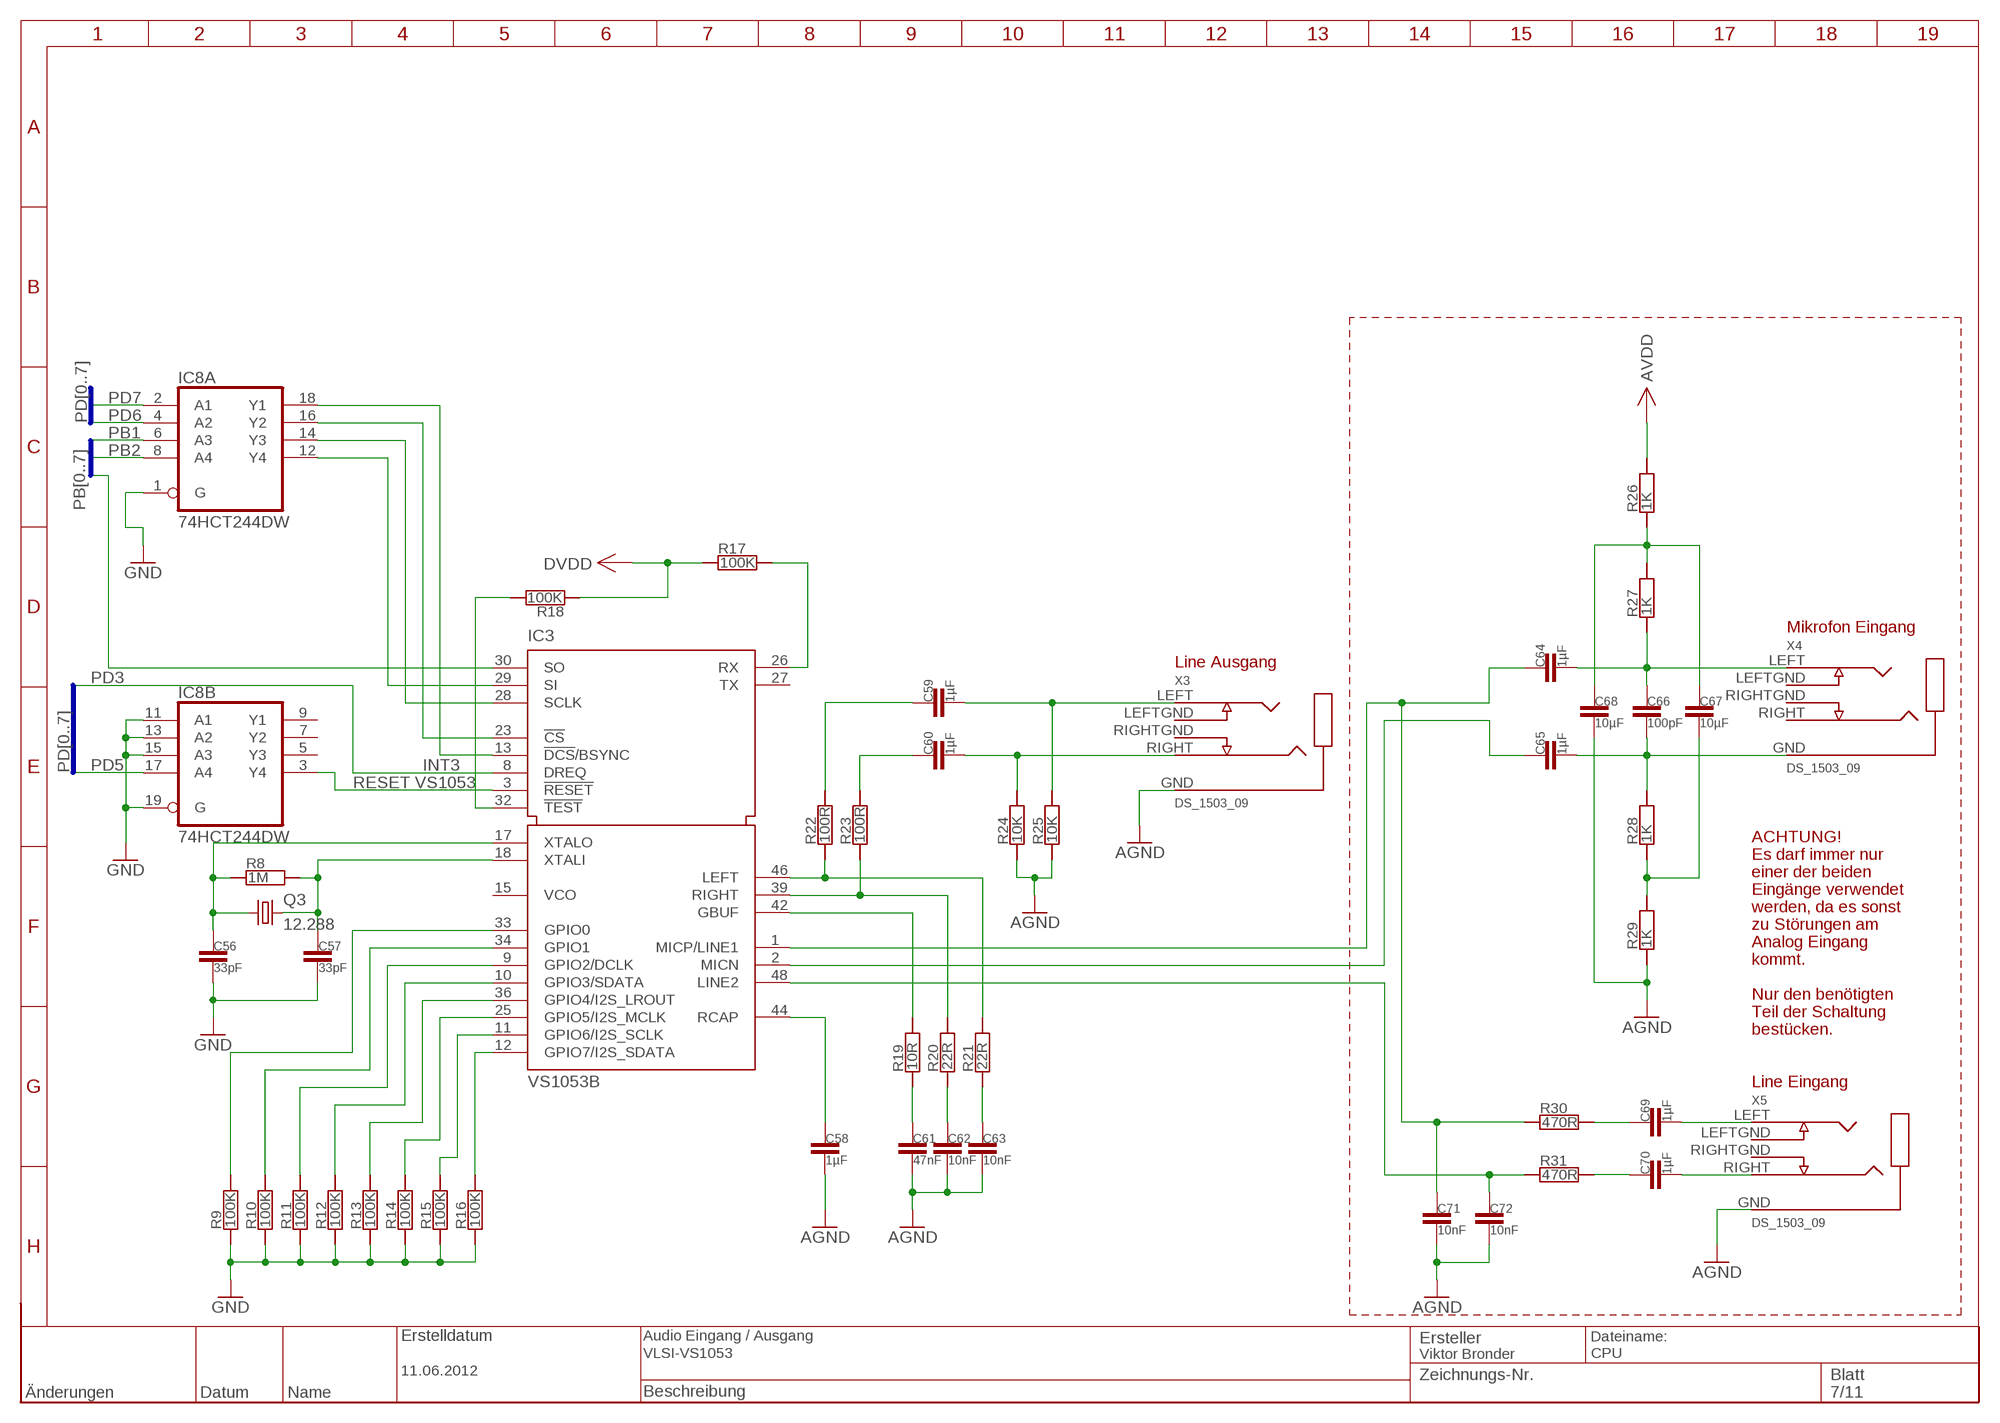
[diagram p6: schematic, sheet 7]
RAHMEN7 (RAHMEN_A4_8Z-19S): BESCHREIBUNG1: Audio Eingang / Ausgang; BESCHREIBUNG2: VLSI-VS1053; ERSTELLDATUM: 11.06.2012; ERSTELLER: Viktor Bronder

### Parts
C56  33pF  C-SMD0603  [0603]
C57  33pF  C-SMD0603  [0603]
C58  1µF  C-SMD0603  [0603]
C59  1µF  C-SMD0603  [0603]
C60  1µF  C-SMD0603  [0603]
C61  47nF  C-SMD  [0805]
C62  10nF  C-SMD0603  [0603]
C63  10nF  C-SMD0603  [0603]
C64  1µF  C-SMD0603  [0603]
C65  1µF  C-SMD0603  [0603]
C66  100pF  C-SMD0603  [0603]
C67  10µF  C-SMD0603  [0603]
C68  10µF  C-SMD0603  [0603]
C69  1µF  C-SMD0603  [0603]
C70  1µF  C-SMD0603  [0603]
C71  10nF  C-SMD0603  [0603]
C72  10nF  C-SMD0603  [0603]
Q3  12.288  CRYSTALHC49U-V  [HC49U-V]
R8  1M  R-SMD0603  [0603]
R9  100K  R-SMD0603  [0603]
R10  100K  R-SMD0603  [0603]
R11  100K  R-SMD0603  [0603]
R12  100K  R-SMD0603  [0603]
R13  100K  R-SMD0603  [0603]
R14  100K  R-SMD0603  [0603]
R15  100K  R-SMD0603  [0603]
R16  100K  R-SMD0603  [0603]
R17  100K  R-SMD0603  [0603]
R18  100K  R-SMD0603  [0603]
R19  10R  R-SMD0603  [0603]
R20  22R  R-SMD0603  [0603]
R21  22R  R-SMD0603  [0603]
R22  100R  R-SMD0603  [0603]
R23  100R  R-SMD0603  [0603]
R24  10K  R-SMD0603  [0603]
R25  10K  R-SMD0603  [0603]
R26  1K  R-SMD0603  [0603]
R27  1K  R-SMD0603  [0603]
R28  1K  R-SMD0603  [0603]
R29  1K  R-SMD0603  [0603]
R30  470R  R-SMD0603  [0603]
R31  470R  R-SMD0603  [0603]
X3  DS_1503_09  [EBS35]
X4  DS_1503_09  [EBS35]
X5  DS_1503_09  [EBS35]

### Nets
AGND: C58.2 C61.2 C62.2 C63.2 C68.2 C71.2 C72.2 R24.1 R25.1 R29.1 X3.GND X5.GND ; also sheet 2,3
AVDD: R26.2 ; also sheet 2,3
DVDD: R17.1 R18.1 ; also sheet 2,3
GND: C56.2 C57.2 IC8.1(A:G) IC8.11(B:A1) IC8.13(B:A2) IC8.15(B:A3) IC8.19(B:G) R9.1 R10.1 R11.1 R12.1 R13.1 R14.1 R15.1 R16.1 ; also sheet 2,3,4,5,10
N$19: IC3.12(GPIO7/I2S_SDATA) R16.2
N$20: IC3.11(GPIO6/I2S_SCLK) R15.2
N$21: IC3.25(GPIO5/I2S_MCLK) R14.2
N$22: IC3.36(GPIO4/I2S_LROUT) R13.2
N$23: IC3.10(GPIO3/SDATA) R12.2
N$24: IC3.9(GPIO2/DCLK) R11.2
N$25: IC3.34(GPIO1) R10.2
N$26: IC3.33(GPIO0) R9.2
N$27: C56.1 IC3.17(XTALO) Q3.1 R8.1
N$28: C57.1 IC3.18(XTALI) Q3.2 R8.2
N$29: IC3.32(!TEST) R18.2
N$30: IC3.26(RX) R17.2
N$31: C58.1 IC3.44(RCAP)
N$32: IC3.46(LEFT) R21.2 R22.1
N$33: IC3.39(RIGHT) R20.2 R23.1
N$34: IC3.42(GBUF) R19.2
N$35: C60.1 R23.2
N$36: C59.1 R22.2
N$37: C60.2 R24.2 X3.RIGHT
N$38: C59.2 R25.2 X3.LEFT
N$39: C61.1 R19.1
N$40: C62.1 R20.1
N$41: C63.1 R21.1
N$42: C64.1 C71.1 IC3.1(MICP/LINE1) R30.1
N$43: C65.1 IC3.2(MICN)
N$44: C64.2 C66.1 R27.1 X4.LEFT
N$45: C65.2 C66.2 R28.2 X4.GND
N$46: C67.2 R28.1 R29.2
N$47: C67.1 C68.1 R26.1 R27.2
N$48: C72.1 IC3.48(LINE2) R31.1
N$49: C69.2 X5.LEFT
N$50: C70.2 X5.RIGHT
N$51: C69.1 R30.2
N$52: C70.1 R31.2
N$53: IC3.23(!CS) IC8.16(A:Y2)
N$57: IC3.13(!DCS!/BSYNC) IC8.18(A:Y1)
N$58: IC3.3(!RESET) IC8.3(B:Y4)
N$59: IC3.29(SI) IC8.12(A:Y4)
N$60: IC3.28(SCLK) IC8.14(A:Y3)
PB1: IC8.6(A:A3) ; also sheet 8,10
PB2: IC8.8(A:A4) ; also sheet 8,10
PB3: IC3.30(SO) ; also sheet 8,10
PD3: IC3.8(DREQ) ; also sheet 8
PD5: IC8.17(B:A4) ; also sheet 8
PD6: IC8.4(A:A2) ; also sheet 8
PD7: IC8.2(A:A1) ; also sheet 8
Unconnected: IC3.15(VCO) IC3.27(TX) IC8.5(B:Y3) IC8.7(B:Y2) IC8.9(B:Y1) X3.LEFTGND X3.RIGHTGND X4.LEFTGND X4.RIGHT X4.RIGHTGND X5.LEFTGND X5.RIGHTGND

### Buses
PB[0..7]
PD[0..7]

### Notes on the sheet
- Mikrofon Eingang
- Line Ausgang
- INT3
- RESET VS1053
- ACHTUNG!
- Es darf immer nur
- einer der beiden
- Eingänge verwendet
- werden, da es sonst
- zu Störungen am
- Analog Eingang
- kommt.
- Nur den benötigten
- Teil der Schaltung
- bestücken.
- Line Eingang

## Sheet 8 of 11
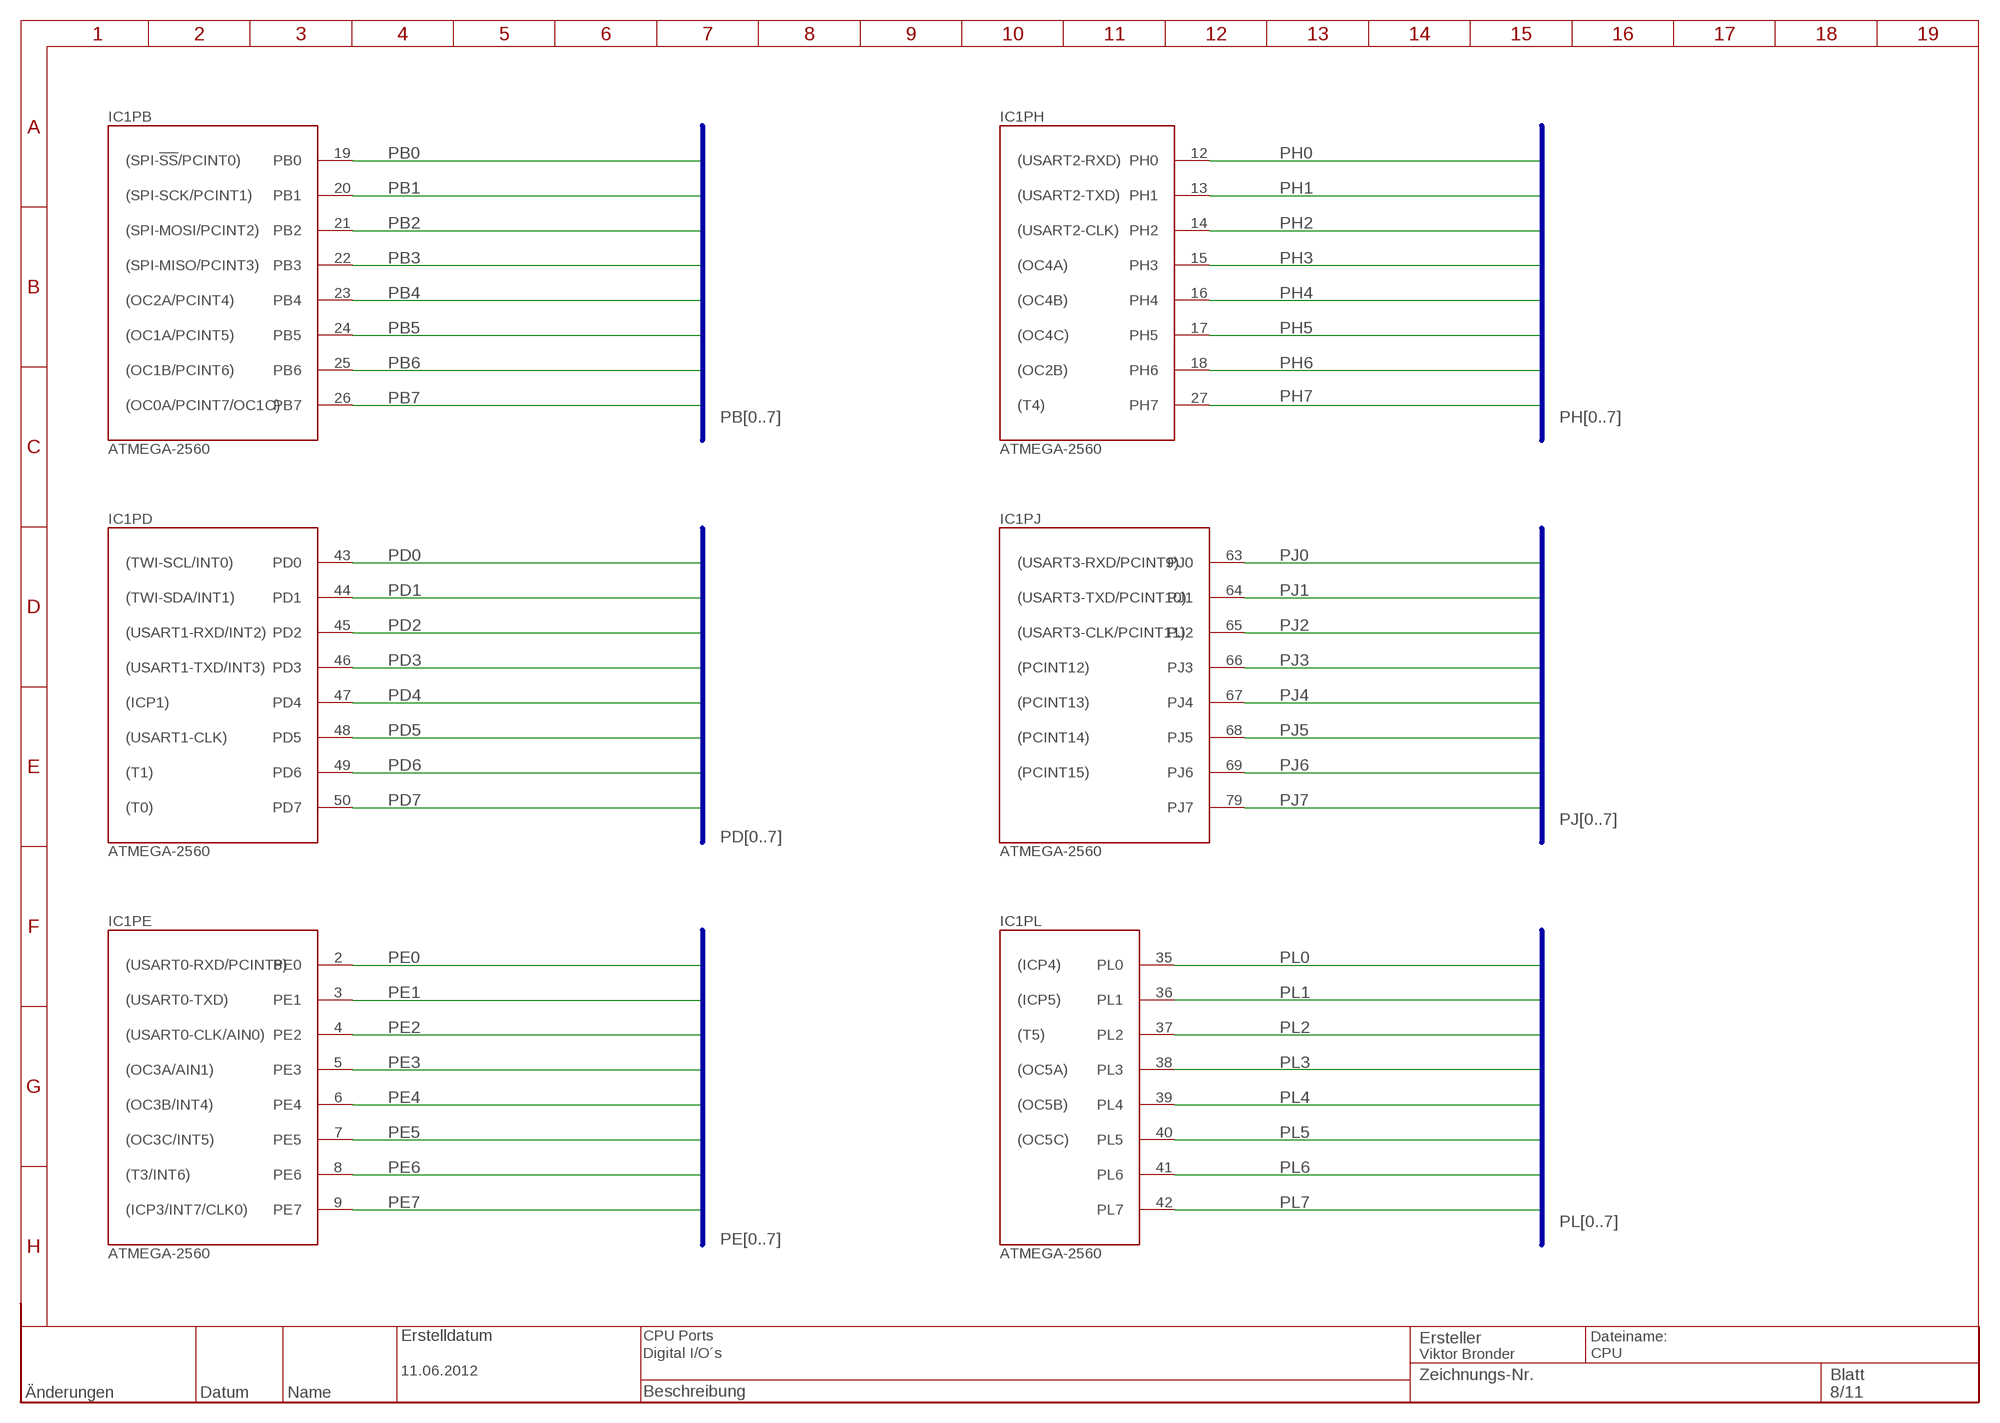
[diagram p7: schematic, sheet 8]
RAHMEN8 (RAHMEN_A4_8Z-19S): BESCHREIBUNG1: CPU Ports; BESCHREIBUNG2: Digital I/O´s; ERSTELLDATUM: 11.06.2012; ERSTELLER: Viktor Bronder

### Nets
PB0: IC1.19(PB:PB0) ; also sheet 10
PB1: IC1.20(PB:PB1) ; also sheet 7,10
PB2: IC1.21(PB:PB2) ; also sheet 7,10
PB3: IC1.22(PB:PB3) ; also sheet 7,10
PB4: IC1.23(PB:PB4) ; also sheet 10
PB5: IC1.24(PB:PB5) ; also sheet 10
PB6: IC1.25(PB:PB6) ; also sheet 10
PB7: IC1.26(PB:PB7) ; also sheet 10
PD0: IC1.43(PD:PD0) ; also sheet 10
PD1: IC1.44(PD:PD1) ; also sheet 10
PD2: IC1.45(PD:PD2) ; also sheet 5
PD3: IC1.46(PD:PD3) ; also sheet 7
PD4: IC1.47(PD:PD4) ; also sheet 5
PD5: IC1.48(PD:PD5) ; also sheet 7
PD6: IC1.49(PD:PD6) ; also sheet 7
PD7: IC1.50(PD:PD7) ; also sheet 7
PE0: IC1.2(PE:PE0) ; also sheet 10
PE1: IC1.3(PE:PE1) ; also sheet 10
PE2: IC1.4(PE:PE2) ; also sheet 10
PE3: IC1.5(PE:PE3) ; also sheet 10
PE4: IC1.6(PE:PE4) ; also sheet 10
PE5: IC1.7(PE:PE5) ; also sheet 10
PE6: IC1.8(PE:PE6) ; also sheet 10
PE7: IC1.9(PE:PE7) ; also sheet 10
PH0: IC1.12(PH:PH0) ; also sheet 10
PH1: IC1.13(PH:PH1) ; also sheet 10
PH2: IC1.14(PH:PH2) ; also sheet 10
PH3: IC1.15(PH:PH3) ; also sheet 10
PH4: IC1.16(PH:PH4) ; also sheet 10
PH5: IC1.17(PH:PH5) ; also sheet 10
PH6: IC1.18(PH:PH6) ; also sheet 10
PH7: IC1.27(PH:PH7) ; also sheet 10
PJ0: IC1.63(PJ:PJ0) ; also sheet 10
PJ1: IC1.64(PJ:PJ1) ; also sheet 10
PJ2: IC1.65(PJ:PJ2) ; also sheet 10
PJ3: IC1.66(PJ:PJ3) ; also sheet 10
PJ4: IC1.67(PJ:PJ4) ; also sheet 10
PJ5: IC1.68(PJ:PJ5) ; also sheet 10
PJ6: IC1.69(PJ:PJ6) ; also sheet 10
PJ7: IC1.79(PJ:PJ7) ; also sheet 10
PL0: IC1.35(PL:PL0) ; also sheet 10
PL1: IC1.36(PL:PL1) ; also sheet 10
PL2: IC1.37(PL:PL2) ; also sheet 10
PL3: IC1.38(PL:PL3) ; also sheet 10
PL4: IC1.39(PL:PL4) ; also sheet 10
PL5: IC1.40(PL:PL5) ; also sheet 10
PL6: IC1.41(PL:PL6) ; also sheet 10
PL7: IC1.42(PL:PL7) ; also sheet 10

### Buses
PB[0..7]
PD[0..7]
PE[0..7]
PH[0..7]
PJ[0..7]
PL[0..7]

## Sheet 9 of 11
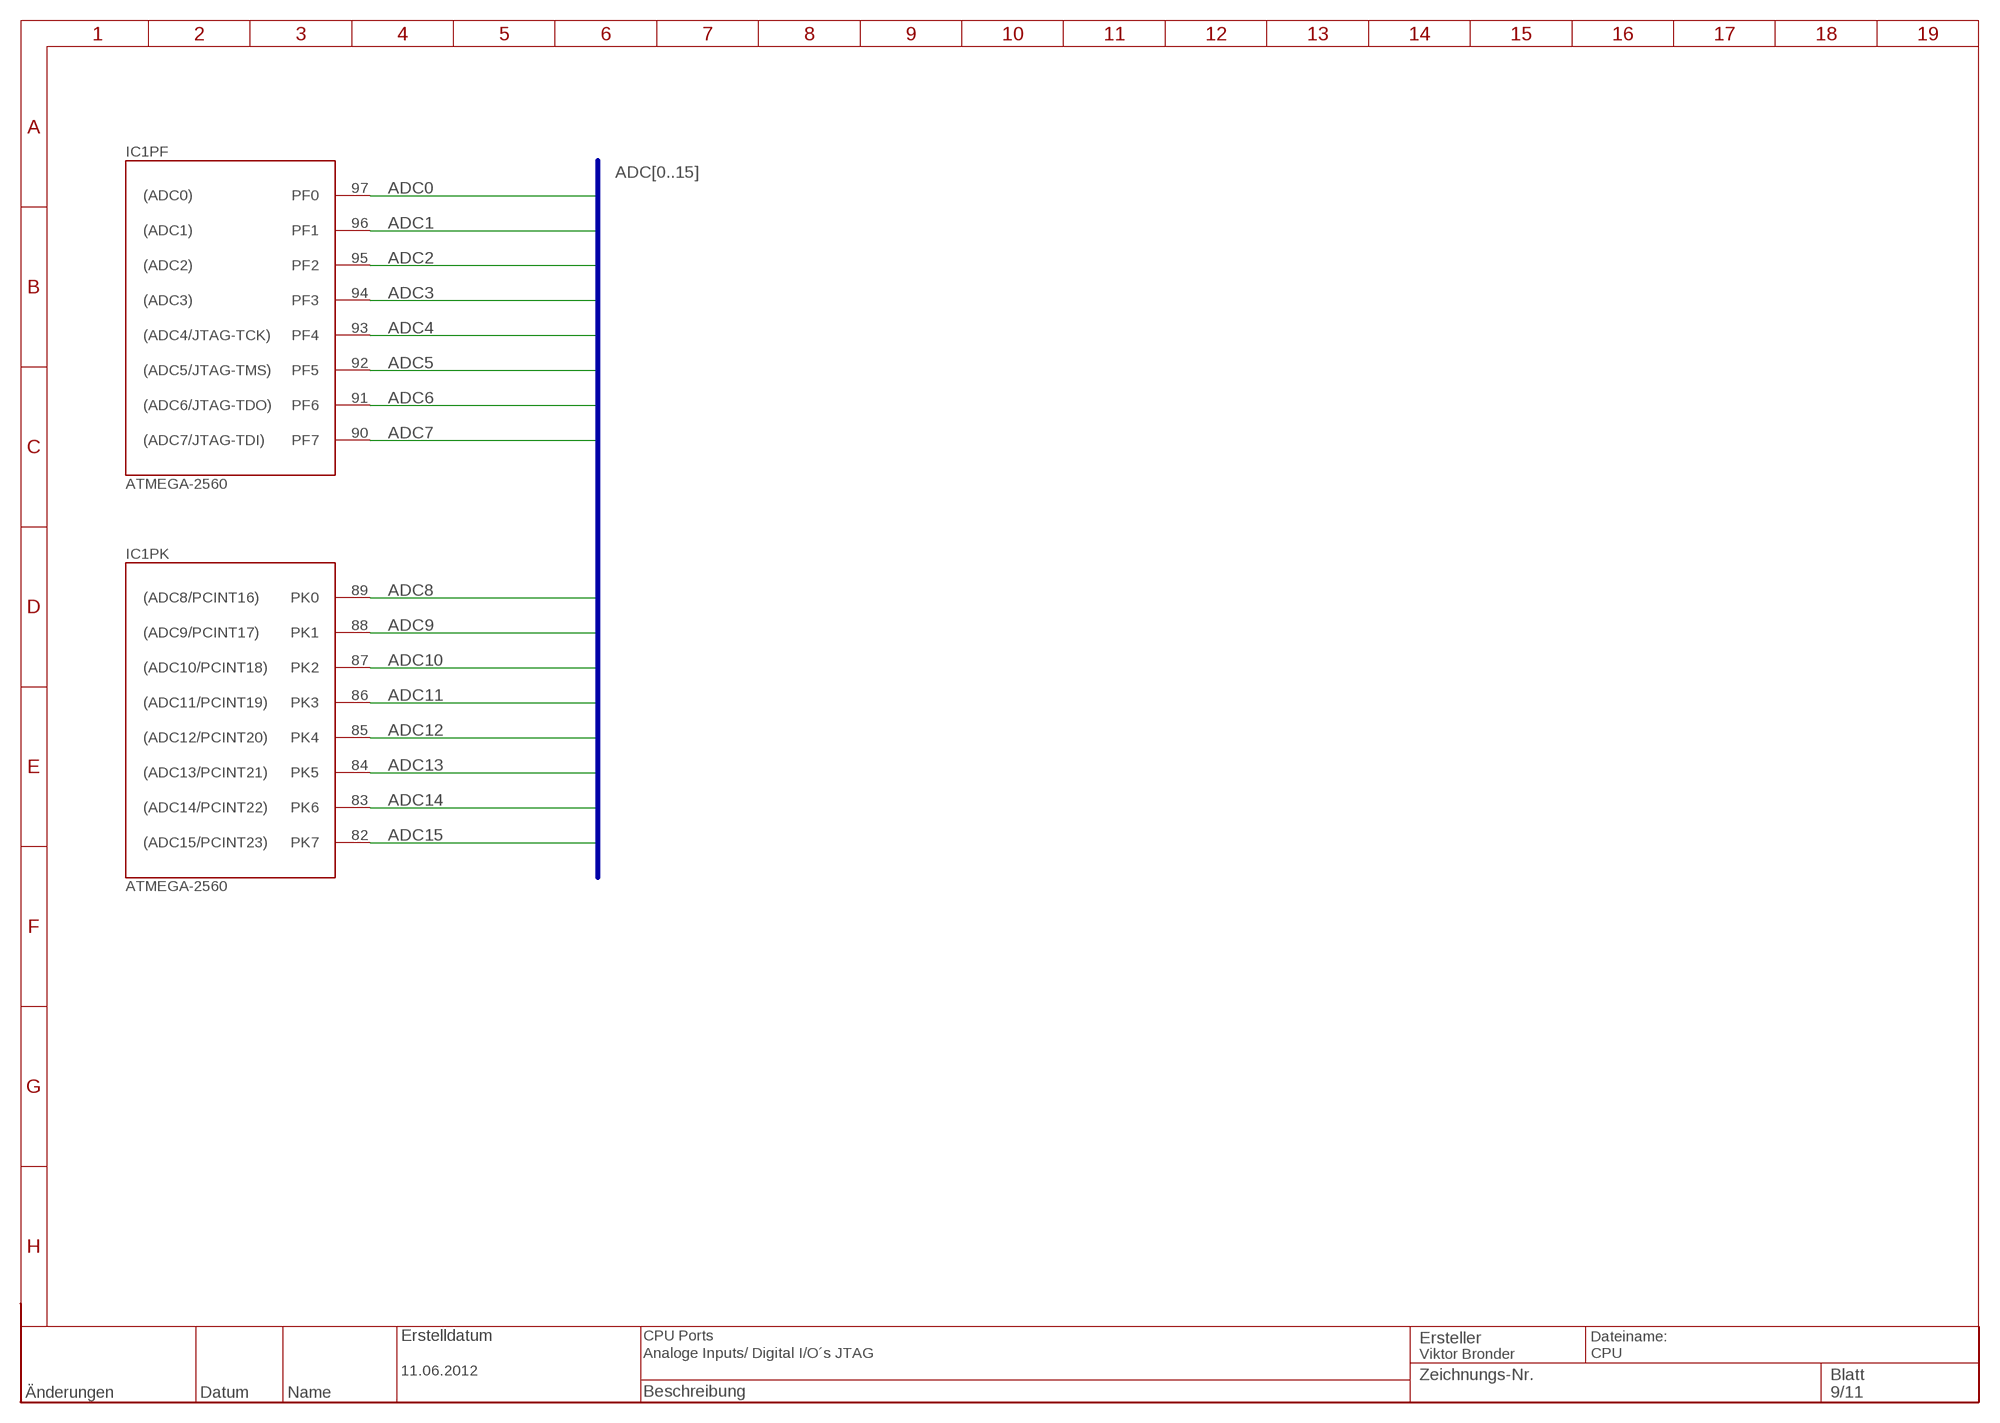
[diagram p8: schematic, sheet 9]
RAHMEN9 (RAHMEN_A4_8Z-19S): BESCHREIBUNG1: CPU Ports; BESCHREIBUNG2: Analoge Inputs/ Digital I/O´s JTAG; ERSTELLDATUM: 11.06.2012; ERSTELLER: Viktor Bronder

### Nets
ADC0: IC1.97(PF:PF0) ; also sheet 10
ADC1: IC1.96(PF:PF1) ; also sheet 10
ADC2: IC1.95(PF:PF2) ; also sheet 10
ADC3: IC1.94(PF:PF3) ; also sheet 10
ADC4: IC1.93(PF:PF4) ; also sheet 10
ADC5: IC1.92(PF:PF5) ; also sheet 10
ADC6: IC1.91(PF:PF6) ; also sheet 10
ADC7: IC1.90(PF:PF7) ; also sheet 10
ADC8: IC1.89(PK:PK0) ; also sheet 10
ADC9: IC1.88(PK:PK1) ; also sheet 10
ADC10: IC1.87(PK:PK2) ; also sheet 10
ADC11: IC1.86(PK:PK3) ; also sheet 10
ADC12: IC1.85(PK:PK4) ; also sheet 10
ADC13: IC1.84(PK:PK5) ; also sheet 10
ADC14: IC1.83(PK:PK6) ; also sheet 10
ADC15: IC1.82(PK:PK7) ; also sheet 10

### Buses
ADC[0..15]

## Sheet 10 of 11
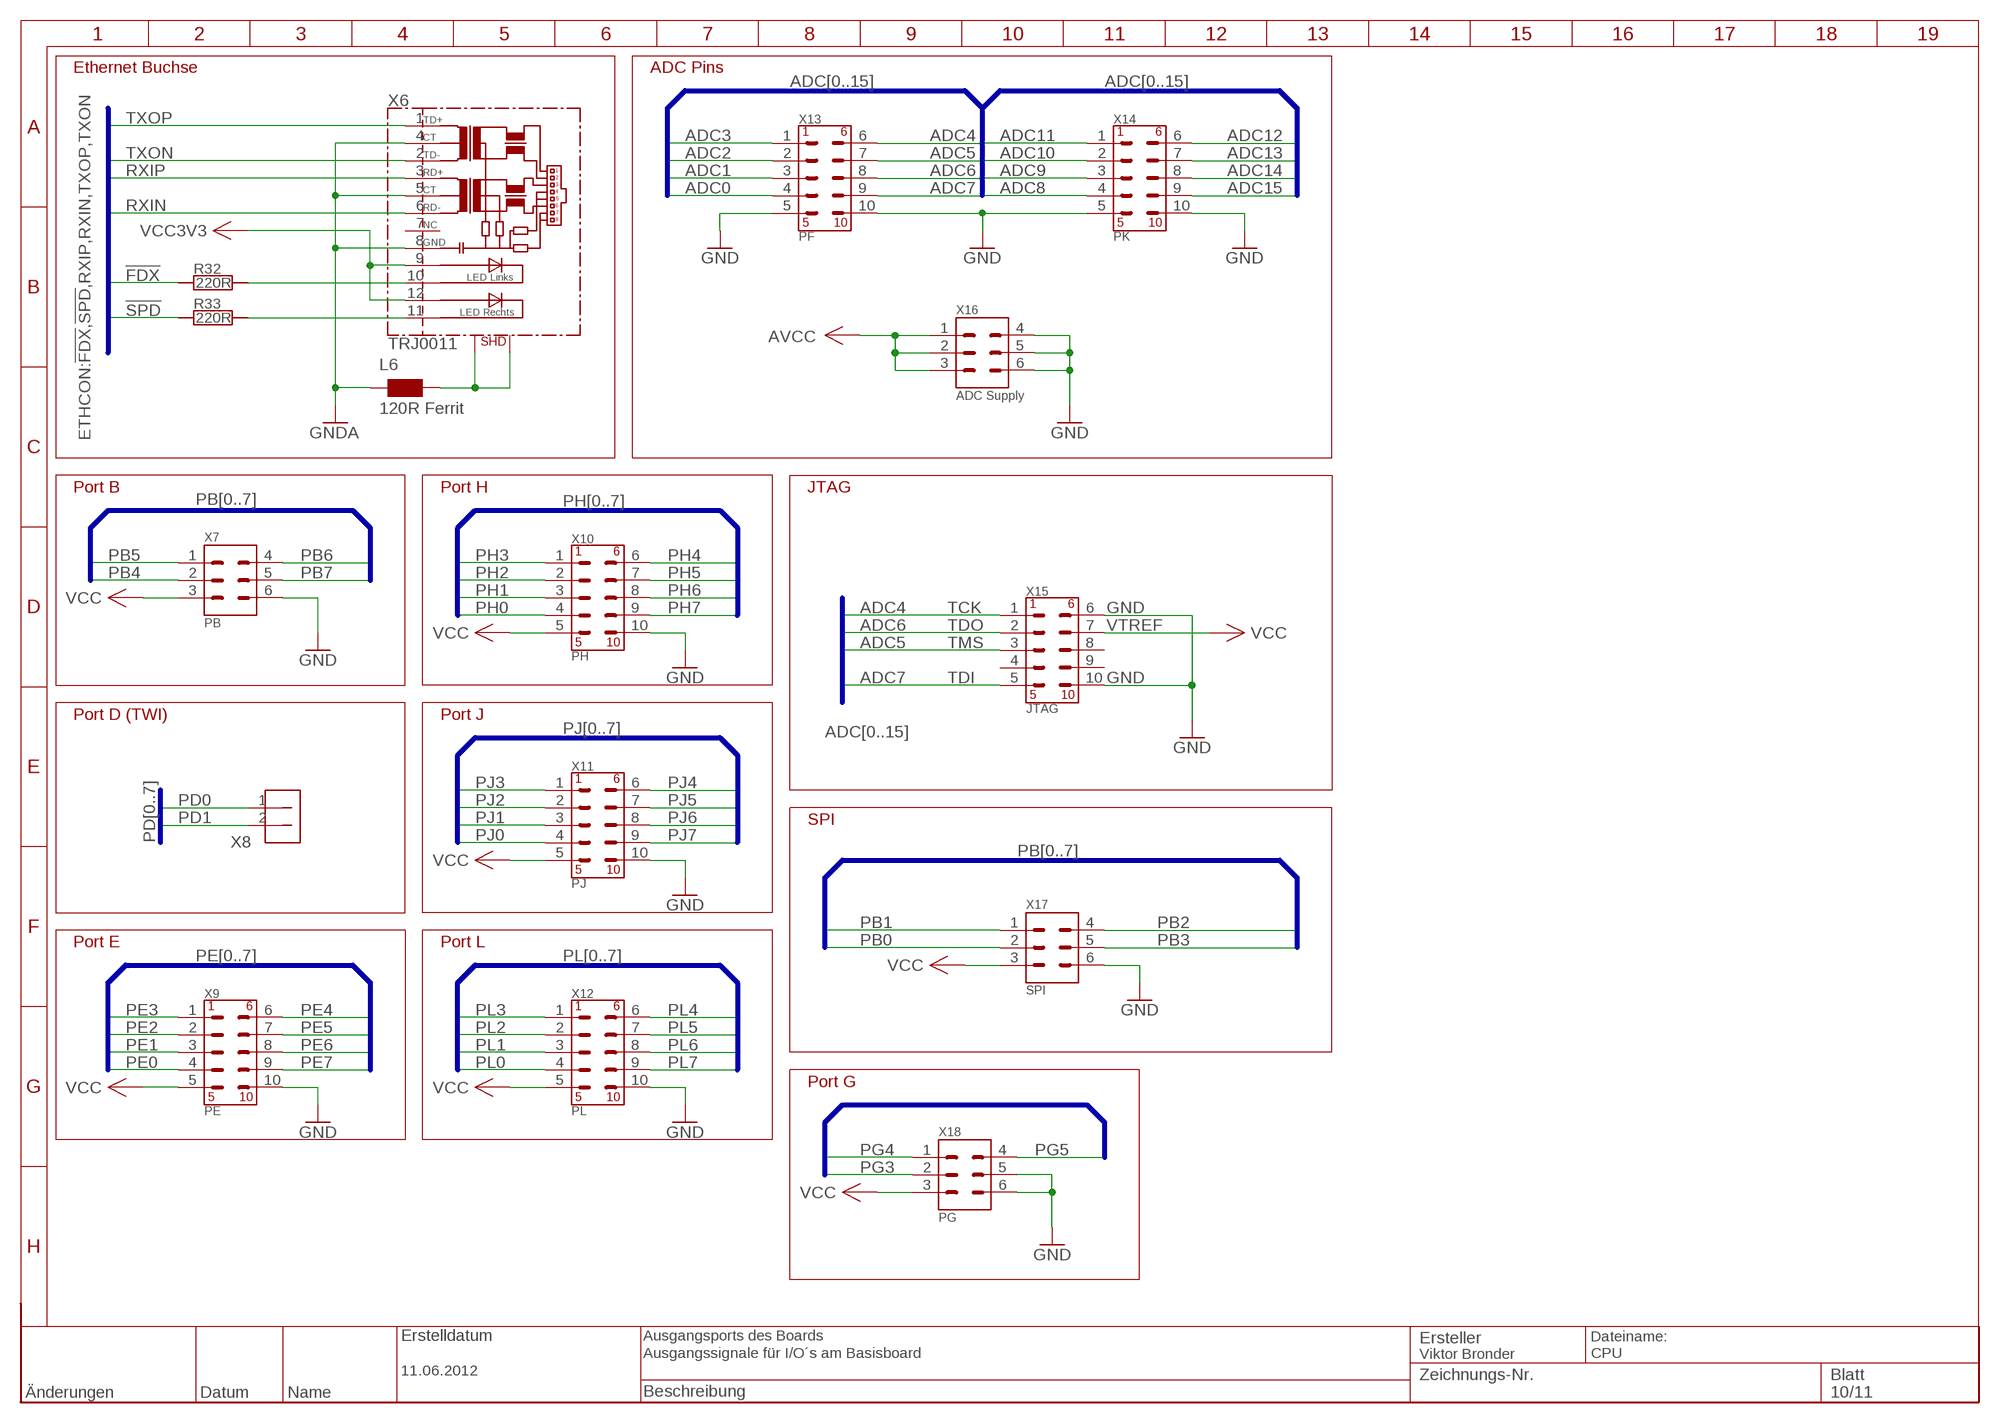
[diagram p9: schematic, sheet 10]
RAHMEN10 (RAHMEN_A4_8Z-19S): BESCHREIBUNG1: Ausgangsports des Boards; BESCHREIBUNG2: Ausgangssignale für I/O´s am Basisboard; ERSTELLDATUM: 11.06.2012; ERSTELLER: Viktor Bronder

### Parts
L6  120R Ferrit  WE-CBF_0805  [0805]
R32  220R  R-SMD0603  [0603]
R33  220R  R-SMD0603  [0603]
X6  TRJ0011  [TRJ0011]
X7  PB  STIFTLEISTE-6PIN  [STIFTLEISTE-2X3PIN]
X8  TWI  STIFTLEISTE-2PIN  [STIFTLEISTE-2PIN]
X9  PE  STIFTLEISTE-10PIN  [STIFTLEISTE-2X5PIN]
X10  PH  STIFTLEISTE-10PIN  [STIFTLEISTE-2X5PIN]
X11  PJ  STIFTLEISTE-10PIN  [STIFTLEISTE-2X5PIN]
X12  PL  STIFTLEISTE-10PIN  [STIFTLEISTE-2X5PIN]
X13  PF  STIFTLEISTE-10PIN  [STIFTLEISTE-2X5PIN]
X14  PK  STIFTLEISTE-10PIN  [STIFTLEISTE-2X5PIN]
X15  JTAG  STIFTLEISTE-10PIN  [STIFTLEISTE-2X5PIN]
X16  ADC Supply  STIFTLEISTE-6PIN  [STIFTLEISTE-2X3PIN]
X17  SPI  STIFTLEISTE-6PIN  [STIFTLEISTE-2X3PIN]
X18  PG  STIFTLEISTE-6PIN  [STIFTLEISTE-2X3PIN]

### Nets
!FDX: R32.1 ; also sheet 5
!SPD: R33.1 ; also sheet 5
ADC0: X13.4 ; also sheet 9
ADC1: X13.3 ; also sheet 9
ADC2: X13.2 ; also sheet 9
ADC3: X13.1 ; also sheet 9
ADC4: X13.6 X15.1 ; also sheet 9
ADC5: X13.7 X15.3 ; also sheet 9
ADC6: X13.8 X15.2 ; also sheet 9
ADC7: X13.9 X15.5 ; also sheet 9
ADC8: X14.4 ; also sheet 9
ADC9: X14.3 ; also sheet 9
ADC10: X14.2 ; also sheet 9
ADC11: X14.1 ; also sheet 9
ADC12: X14.6 ; also sheet 9
ADC13: X14.7 ; also sheet 9
ADC14: X14.8 ; also sheet 9
ADC15: X14.9 ; also sheet 9
AVCC: X16.1 X16.2 X16.3 ; also sheet 2,3
GND: X7.6 X9.10 X10.10 X11.10 X12.10 X13.5 X13.10 X14.5 X14.10 X15.6 X15.10 X16.4 X16.5 X16.6 X17.6 X18.5 X18.6 ; also sheet 2,3,4,5,7
GNDA: L6.1 X6.4(CTT) X6.5(CTR) X6.8(CHSGND) ; also sheet 2,5
N$54: R32.2 X6.10(LEDL-)
N$55: R33.2 X6.11(LEDR-)
N$56: L6.2 X6.SHD@0(SHD) X6.SHD@1(SHD)
PB0: X17.2 ; also sheet 8
PB1: X17.1 ; also sheet 7,8
PB2: X17.4 ; also sheet 7,8
PB3: X17.5 ; also sheet 7,8
PB4: X7.2 ; also sheet 8
PB5: X7.1 ; also sheet 8
PB6: X7.4 ; also sheet 8
PB7: X7.5 ; also sheet 8
PD0: X8.1 ; also sheet 8
PD1: X8.2 ; also sheet 8
PE0: X9.4 ; also sheet 8
PE1: X9.3 ; also sheet 8
PE2: X9.2 ; also sheet 8
PE3: X9.1 ; also sheet 8
PE4: X9.6 ; also sheet 8
PE5: X9.7 ; also sheet 8
PE6: X9.8 ; also sheet 8
PE7: X9.9 ; also sheet 8
PG3: X18.2 ; also sheet 4
PG4: X18.1 ; also sheet 4
PG5: X18.4 ; also sheet 4
PH0: X10.4 ; also sheet 8
PH1: X10.3 ; also sheet 8
PH2: X10.2 ; also sheet 8
PH3: X10.1 ; also sheet 8
PH4: X10.6 ; also sheet 8
PH5: X10.7 ; also sheet 8
PH6: X10.8 ; also sheet 8
PH7: X10.9 ; also sheet 8
PJ0: X11.4 ; also sheet 8
PJ1: X11.3 ; also sheet 8
PJ2: X11.2 ; also sheet 8
PJ3: X11.1 ; also sheet 8
PJ4: X11.6 ; also sheet 8
PJ5: X11.7 ; also sheet 8
PJ6: X11.8 ; also sheet 8
PJ7: X11.9 ; also sheet 8
PL0: X12.4 ; also sheet 8
PL1: X12.3 ; also sheet 8
PL2: X12.2 ; also sheet 8
PL3: X12.1 ; also sheet 8
PL4: X12.6 ; also sheet 8
PL5: X12.7 ; also sheet 8
PL6: X12.8 ; also sheet 8
PL7: X12.9 ; also sheet 8
RXIN: X6.6(RD-) ; also sheet 5
RXIP: X6.3(RD+) ; also sheet 5
TXON: X6.2(TD-) ; also sheet 5
TXOP: X6.1(TD+) ; also sheet 5
VCC: X7.3 X9.5 X10.5 X11.5 X12.5 X15.7 X17.3 X18.3 ; also sheet 2,3
VCC3V3: X6.9(LEDL+) X6.12(LEDR+) ; also sheet 2,3,5
Unconnected: X6.7(NC) X15.4 X15.8 X15.9

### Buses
ETHCON:!FDX,!SPD,RXIP,RXIN,TXOP,TXON
PB[0..7]
PD[0..7]
PE[0..7]
PH[0..7]
PJ[0..7]
PL[0..7]
ADC[0..15]
PG[3..5]

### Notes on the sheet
- Ethernet Buchse | ADC Pins
- Port B | Port H | JTAG
- TCK | GND
- TDO | VTREF
- TMS
- TDI | GND
- Port D (TWI) | Port J
- SPI
- Port E | Port L
- Port G

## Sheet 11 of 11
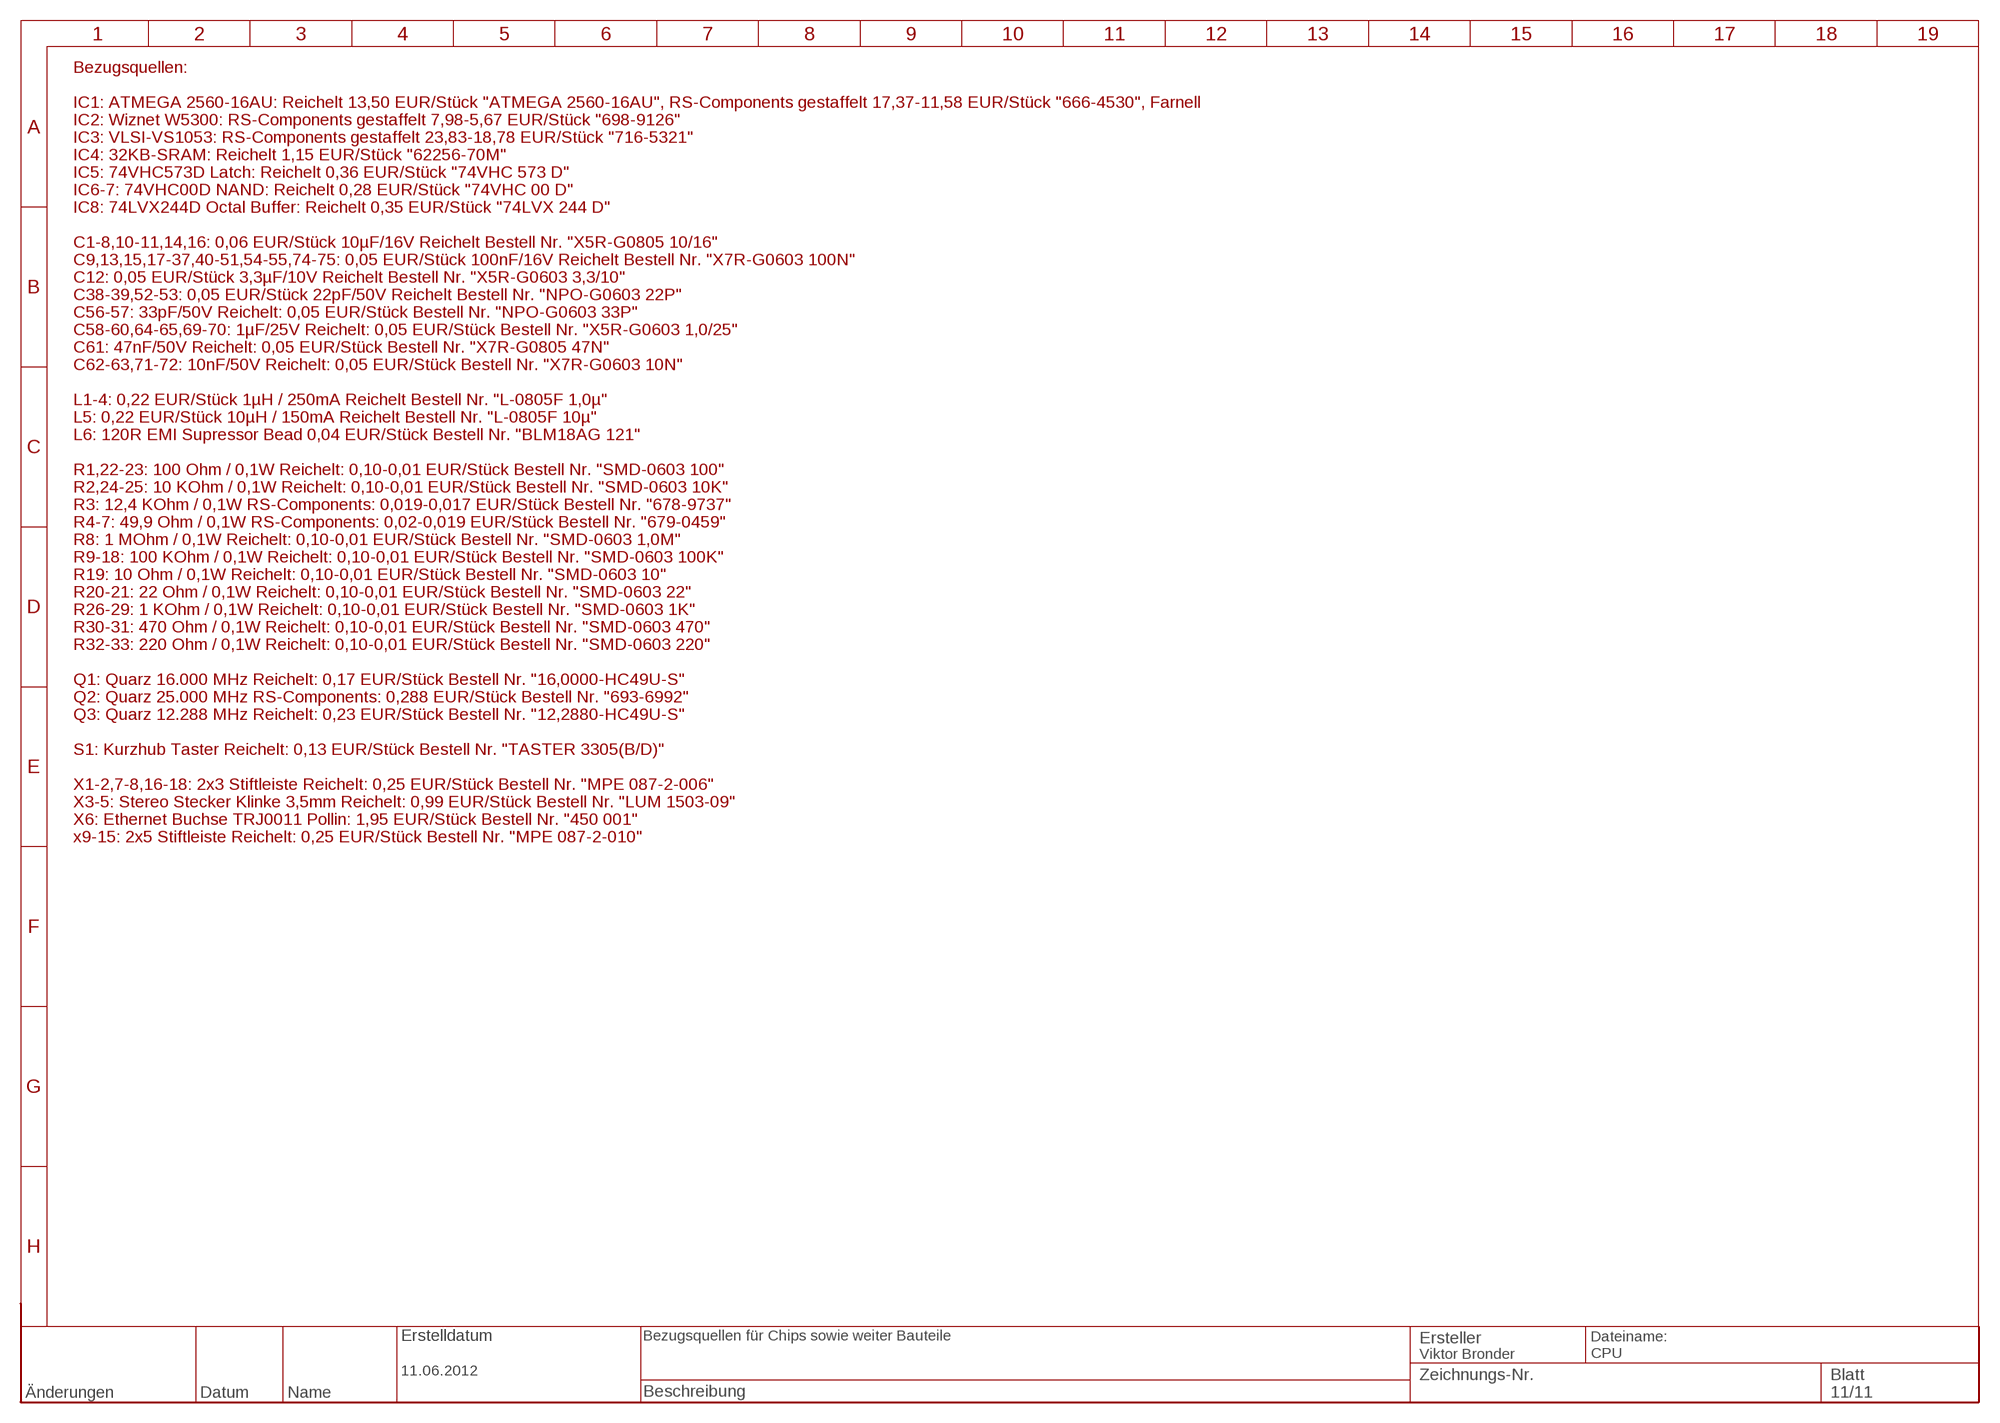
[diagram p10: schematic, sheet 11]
RAHMEN11 (RAHMEN_A4_8Z-19S): BESCHREIBUNG1: Bezugsquellen für Chips sowie weiter Bauteile; ERSTELLDATUM: 11.06.2012; ERSTELLER: Viktor Bronder

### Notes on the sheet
- Bezugsquellen:
- IC1: ATMEGA 2560-16AU: Reichelt 13,50 EUR/Stück "ATMEGA 2560-16AU", RS-Components gestaffelt 17,37-11,58 EUR/Stück "666-4530", Farnell
- IC2: Wiznet W5300: RS-Components gestaffelt 7,98-5,67 EUR/Stück "698-9126"
- IC3: VLSI-VS1053: RS-Components gestaffelt 23,83-18,78 EUR/Stück "716-5321"
- IC4: 32KB-SRAM: Reichelt 1,15 EUR/Stück "62256-70M"
- IC5: 74VHC573D Latch: Reichelt 0,36 EUR/Stück "74VHC 573 D"
- IC6-7: 74VHC00D NAND: Reichelt 0,28 EUR/Stück "74VHC 00 D"
- IC8: 74LVX244D Octal Buffer: Reichelt 0,35 EUR/Stück "74LVX 244 D"
- C1-8,10-11,14,16: 0,06 EUR/Stück 10µF/16V Reichelt Bestell Nr. "X5R-G0805 10/16"
- C9,13,15,17-37,40-51,54-55,74-75: 0,05 EUR/Stück 100nF/16V Reichelt Bestell Nr. "X7R-G0603 100N"
- C12: 0,05 EUR/Stück 3,3µF/10V Reichelt Bestell Nr. "X5R-G0603 3,3/10"
- C38-39,52-53: 0,05 EUR/Stück 22pF/50V Reichelt Bestell Nr. "NPO-G0603 22P"
- C56-57: 33pF/50V Reichelt: 0,05 EUR/Stück Bestell Nr. "NPO-G0603 33P"
- C58-60,64-65,69-70: 1µF/25V Reichelt: 0,05 EUR/Stück Bestell Nr. "X5R-G0603 1,0/25"
- C61: 47nF/50V Reichelt: 0,05 EUR/Stück Bestell Nr. "X7R-G0805 47N"
- C62-63,71-72: 10nF/50V Reichelt: 0,05 EUR/Stück Bestell Nr. "X7R-G0603 10N"
- L1-4: 0,22 EUR/Stück 1µH / 250mA Reichelt Bestell Nr. "L-0805F 1,0µ"
- L5: 0,22 EUR/Stück 10µH / 150mA Reichelt Bestell Nr. "L-0805F 10µ"
- L6: 120R EMI Supressor Bead 0,04 EUR/Stück Bestell Nr. "BLM18AG 121"
- R1,22-23: 100 Ohm / 0,1W Reichelt: 0,10-0,01 EUR/Stück Bestell Nr. "SMD-0603 100"
- R2,24-25: 10 KOhm / 0,1W Reichelt: 0,10-0,01 EUR/Stück Bestell Nr. "SMD-0603 10K"
- R3: 12,4 KOhm / 0,1W RS-Components: 0,019-0,017 EUR/Stück Bestell Nr. "678-9737"
- R4-7: 49,9 Ohm / 0,1W RS-Components: 0,02-0,019 EUR/Stück Bestell Nr. "679-0459"
- R8: 1 MOhm / 0,1W Reichelt: 0,10-0,01 EUR/Stück Bestell Nr. "SMD-0603 1,0M"
- R9-18: 100 KOhm / 0,1W Reichelt: 0,10-0,01 EUR/Stück Bestell Nr. "SMD-0603 100K"
- R19: 10 Ohm / 0,1W Reichelt: 0,10-0,01 EUR/Stück Bestell Nr. "SMD-0603 10"
- R20-21: 22 Ohm / 0,1W Reichelt: 0,10-0,01 EUR/Stück Bestell Nr. "SMD-0603 22"
- R26-29: 1 KOhm / 0,1W Reichelt: 0,10-0,01 EUR/Stück Bestell Nr. "SMD-0603 1K"
- R30-31: 470 Ohm / 0,1W Reichelt: 0,10-0,01 EUR/Stück Bestell Nr. "SMD-0603 470"
- R32-33: 220 Ohm / 0,1W Reichelt: 0,10-0,01 EUR/Stück Bestell Nr. "SMD-0603 220"
- Q1: Quarz 16.000 MHz Reichelt: 0,17 EUR/Stück Bestell Nr. "16,0000-HC49U-S"
- Q2: Quarz 25.000 MHz RS-Components: 0,288 EUR/Stück Bestell Nr. "693-6992"
- Q3: Quarz 12.288 MHz Reichelt: 0,23 EUR/Stück Bestell Nr. "12,2880-HC49U-S"
- S1: Kurzhub Taster Reichelt: 0,13 EUR/Stück Bestell Nr. "TASTER 3305(B/D)"
- X1-2,7-8,16-18: 2x3 Stiftleiste Reichelt: 0,25 EUR/Stück Bestell Nr. "MPE 087-2-006"
- X3-5: Stereo Stecker Klinke 3,5mm Reichelt: 0,99 EUR/Stück Bestell Nr. "LUM 1503-09"
- X6: Ethernet Buchse TRJ0011 Pollin: 1,95 EUR/Stück Bestell Nr. "450 001"
- x9-15: 2x5 Stiftleiste Reichelt: 0,25 EUR/Stück Bestell Nr. "MPE 087-2-010"

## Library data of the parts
BR1-BR9 = Versorgungssymbole:0-OHM-BRÜCKE: ACHTUNG
C1-C75 = Kondensator:C-SMD
IC1 = Mikrocontroller:ATMEGA-2560
IC2 = Mikrocontroller:WIZNET-W5300: WIZNET-W5300 - Supports hardwired TCP/IP protocols : TCP,UDP, ICMP, IPv4, ARP, IGMPv2, PPPoE, Ethernet - Supports 8 independent SOCKETs simultaneously - High network performance : Up to 50Mbps - Supports hybrid TCP/IP stack(software and hardware TCP/IP stack) - Supports PPPoE connection (with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
IC3 = Mikrocontroller:VLSI-VS1053B
IC4 = memory:TC55257DF: MEMORY
IC5 = 74xx-eu:74*573: 8-bit D latch BUS DRIVER
IC6 IC7 = 74xx-eu:74*00: Quad 2-input NAND gate
IC8 = 74xx-eu:74*244: Octal BUFFER and LINE DRIVER, 3-state
L1-L6 = wuerth-elektronik:WE-CBF: SMD EMI Suppression Ferrite Beads
Q1-Q3 = crystal:CRYSTAL: CRYSTAL; OC_FARNELL: 1666969; OC_NEWARK: unknown
R1-R33 = Widerstand:R-SMD: SMD Widerstand
S1 = Schalter-Taster:PHAP3305: Reichelt Bestellnummer: TASTER 3305 3,1mm Pin bis Taste 0,16 Euro TASTER 3305B 8,4mm Pin bis Taste 0,16 Euro TASTER 3305D 11,9mm Pin bis Taste 0,18 Euro Hub 0,25mm 50mA@12V
X1 X2 X7 X16-X18 = Stecker:STIFTLEISTE-6PIN: Stiftleiste/Buchsenleiste doppelreihig 6 pin
X3-X5 = Stecker:DS_1503_09: Reichelt Bestellnummer: LUM 1503-09 3,5mm Klinke Buchse
X6 = Stecker:TRJ0011
X8 = Stecker:STIFTLEISTE-2PIN
X9-X15 = Stecker:STIFTLEISTE-10PIN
